(* Logix 5000 Rung export; software revision 16.04 *)

MODULES
   Local : vendor None type None code None
   MVI56E_AFC : vendor None type None code None
END_MODULES

TYPE AFCEProveProcess :   // Prove process output from processor to the module
STRUCT
   Sequencing : AFCEProveSequencing;   // Prover sequencing
   Temperature : REAL;   // Temperature for Single Probe provers. And Inlet Temperature for Dual Probe Provers.
   OutletTemperature : REAL;   // Outlet Temperature for Provers with Dual Probes.
   SwitchBarTemperature : REAL;   // Switch bar temperature
   Pressure : REAL;   // Pressure for Single Probe provers. And Inlet Pressure for Dual Probe Provers.
   OutletPressure : REAL;   // Outlet Pressure for Provers with Dual Probes.
   ProverDensity : REAL;   // Prover density
END_STRUCT
END_TYPE

TYPE AFCEModbusMasterDataType :   // Modbus master data type
STRUCT
   Bit : BOOL;   // bit type
   Word : BOOL;   // word type (16-bit)
   Long : BOOL;   // long integer (32-bit)
   LongRemote : BOOL;   // long integer (32-bit)
END_STRUCT
END_TYPE

TYPE AFCEProveSequencing :   // AFC prove sequencing tag for phase selection and ball positioning
STRUCT
   Phase : AFCEProvePhaseBitmap;   // AFC phase sequencing
   BallPositionReady : BOOL;   // Ball position: Ready (Udir & Bdir only; fwd leg Bdir)
   BallPositionSealed : BOOL;   // Ball position: Sealed (Udir & Bdir only; fwd leg Bdir)
   BallPositionReadyBwdLeg : BOOL;   // Ball position: Ready bwd leg (Bdir only)
   BallPositionSealedBwdLeg : BOOL;   // Ball position: Sealed bwd leg (Bdir only)
END_STRUCT
END_TYPE

TYPE AFCEUtil :   // Used for internal ladder logic usage. These values must not be changed by user application.
STRUCT
   Flags : AFCEFlag;   // Wallclock update commands
   CycleCounter : INT;   // Reflects current block ID calculated by ladder to be sent to the module
   Buffer : AFCEUtilBuffer;
   Block : AFCEUtilBlock;
END_STRUCT
END_TYPE

TYPE AFCEModbusGatewayCommand :   // Modbus Gateway Command
STRUCT
   Config : AFCEModbusGatewayConfig;   // Config data to be entered by the user.
   Trigger : BOOL;   // Trigger the Command, when cleared module has responded.
   Data : INT[200];   // Contains modbus data written to the module (write commands)
END_STRUCT
END_TYPE

TYPE AFCEProveRunResults :   // Run results of the prove. Copied from the module to the pocessor
STRUCT
   CountAttempted : INT;   // Run count attempted
   CountCompleted : INT;   // Run count completed
   CountSelected : INT;   // Run count selected
   RunsSelected : INT;   // Bit Mapped Runs selected for calculations from completed runs
   NewMeterFactor : REAL;   // New meter factor
   ChangeInMeterFactor : REAL;   // Change in meter factor
END_STRUCT
END_TYPE

TYPE AFCEModbusMasterSwap :   // Modbus master swap words/ swap bytes
STRUCT
   SwapWords : BOOL;   // Swap words
   SwapBytes : BOOL;   // Swap bytes
END_STRUCT
END_TYPE

TYPE AFCEModbusMaster :   // Modbus Master. Port 3 must be configured as modbus master through AFC Manager to use this feature.
STRUCT
   Enable : BOOL;   // Enable the modbus master funcionality
   CommandIndex : INT;   // Selects which command index will be executed
   Command : AFCEModbusMasterCommand[10];   // Each command contains a specific modbus request to be sent out of the port
END_STRUCT
END_TYPE

TYPE AFCEFlag :   // Flags contains status information updated by ladder and also trigger bits for clock update
STRUCT
   AFCStopped : BOOL;   // Indicates that the module has sent a new input block to be processed by ladder - UPDATED BY LADDER
   AFCInputSequenceNum : INT;   // Meter number (0 -15) associated to blocks 1-16. Used to update "Profile" (meter type and product group.) UPDATED BY LADDER
END_STRUCT
END_TYPE

TYPE AFCEModbusPassThruBitData :   // AFC Modbus Pass-thru Bit Data
STRUCT
   Data : BOOL[2016];   // Contains received data for bit commands
END_STRUCT
END_TYPE

TYPE AFCEUtilBlockInterrupt :
STRUCT
   Now : BOOL;
   ModbusGateway : DINT;
   EnableDisable : BOOL;
   Analysis : DINT;
END_STRUCT
END_TYPE

TYPE AFCEFirmwareVersion :
STRUCT
   Major : SINT;   // Major Version number
   Minor : SINT;   // Minor Version number
   Revision : INT;   // Revision
END_STRUCT
END_TYPE

TYPE AFCEModbusGateway :   // Modbus Gateway
STRUCT
   Command : AFCEModbusGatewayCommand[10];   // Modbus gateway commands - contains setup and modbus data
END_STRUCT
END_TYPE

TYPE AFCEUtilBuffer :   // Buffer
STRUCT
   Input : INT[250];   // Input buffer contains the complete block to be copied from the module
   Output : INT[248];   // Output buffer contains data the complete block to be copied to the module
   Process : INT[240];
   ArchiveDay : INT[98];
   ArchiveHour : INT[98];
   Prove : INT[26];
   Analysis : INT[198];
   MeterEnableDisable : INT[4];
   StreamEnable : INT[48];
   StreamDisable : INT[48];
   StreamSelect : INT[32];
   MeterSignals : INT[32];
   Calibration : INT[36];
END_STRUCT
END_TYPE

TYPE AFCEUtilBlock :
STRUCT
   ProcessInput : INT;
   InterruptPending : AFCEUtilBlockInterrupt;
   InterruptComplete : AFCEUtilBlockInterrupt;
   NonInterruptPending : AFCEUtilBlockNonInterrupt;
   NonInterruptComplete : AFCEUtilBlockNonInterrupt;
END_STRUCT
END_TYPE

TYPE AFCEProve :   // Prove
STRUCT
   Process : AFCEProveProcess;   // Process Variables
   Signals : AFCEProveSignals;   // AFC Prove Signals (triggers the proving update)
   Config : AFCEProveConfig;   // AFC Prove Control (configuration settings)
   PulseCounts : AFCEProvePulseCount;   // Pulse counts to be updated at the end of the run/pass
   ConfigInput : AFCEProveInputConfig;   // AFC prover input configuration
   Status : AFCEProveStatus;   // AFC prover status
   ErrorCode : INT;   // Prove error code
   ProveControlsEcho : INT;   // AFC module Echos the state of the Prove Controls
   RequestedMeterEcho : INT;   // AFC module Echos the Meter number requested
   RequestedCurvePointEcho : INT;   // AFC module Echos the requested Curve Point
   RunResults : AFCEProveRunResults;   // Prove and run results
   ProveEnabled : BOOL;   // ON if prove is enabled. This flag is coped from inputbuffer[247]
END_STRUCT
END_TYPE

TYPE AFCEProveConfig :   // Controls (configuration settings) associated to the prover
STRUCT
   Enable : AFCEProveConfigEnable;   // Controls at enable
   Accept : AFCEProveConfigAccept;   // Controls at accept
END_STRUCT
END_TYPE

TYPE AFCEWallclock :
STRUCT
   GetAFCTime : BOOL;   // Get current AFC Time
   SetAFCTimeFromPLCTime : BOOL;   // Set AFC time from PLC time. Updates current AFC time
   EnableLocalDateTime : BOOL;   // Enable Local Date Time.
   AFCTime : AFCETime;   // Coordinated Universal Time. Updated by either getting or setting AFC time.
END_STRUCT
END_TYPE

TYPE AFCEModbusMasterConfig :   // Modbus master command settings
STRUCT
   Enable : BOOL;   // Set to 1 to enable command (0=disable)
   FunctionType : BOOL;   // Set to 1 to select write command (0=read command)
   RegisterBank : BOOL;   // Set to 1 to select input register (0=holding register)
   DataType : AFCEModbusMasterDataType;   // Select data type format
   SwapOption : AFCEModbusMasterSwap;   // Select byte and word swap (1 = swap, 0 = no swap)
   TypeSwap : INT;   // This value is calculated by ladder logic and must not be modified by user
   SlaveAddress : INT;   // Modbus slave address of remote device
   ModbusAddress : INT;   // Modbus data address on remote slave
   ElementCount : INT;   // Number of data elements (125 words)
   TransactionID : INT;   // Transaction ID. This value is returned to the ReturnedTransaction ID when the response has been received.
END_STRUCT
END_TYPE

TYPE AFCESiteStatus :   // Site status bits - contains general information about the module - not meter specific
STRUCT
   AFCActive : BOOL;   // AFC active
   ChecksumAlarms : BOOL;   // Checkum alarm active
   Reserved2 : BOOL;
   Reserved3 : BOOL;
   PLCHalted : BOOL;   // PLC in program mode or missing
   CfgChanged : BOOL;   // Configuration changed
   Powerup : BOOL;   // Module powered up
   ColdStart : BOOL;   // Module performed cold start (BBRAM initialized)
   ModbusMasterPending : BOOL;   // Modbus Master Poll Pending
   ModbusMasterComplete : BOOL;   // Modbus Master Poll Complete
   ModbusPassThruPending : BOOL;   // Modbus Pass-thru Input Pending
   CalibrationRequest : BOOL;   // Calibration request from module
   ProverEnabled : BOOL;   // Prover Enabled
   Reserved13 : BOOL;
   Reserved14 : BOOL;
   Reserved15 : BOOL;
END_STRUCT
END_TYPE

TYPE AFCEModuleDef :   // Main user defined data type
STRUCT
   ModbusGateway : AFCEModbusGateway;   // Reads and write data between processor and module modbus table
   ModbusMaster : AFCEModbusMaster;   // Setup modbus master commands to be sent to remote slaves (through Port 3)
   ModbusPassThru : AFCEModbusPassThru;   // Modbus pass-thru data
   SiteStatus : AFCESiteStatus;   // Site status
   MeterAlarms : AFCESiteAlarms;   // Meter Alarms
   Prove : AFCEProve;   // Prover
   Wallclock : AFCEWallclock;   // Set clock and get clock information
   Firmware : AFCEFirmwareVersion;   // Firmware information
   Util : AFCEUtil;   // Used by ladder logic
END_STRUCT
END_TYPE

TYPE AFCEModbusGatewayConfig :   // Modbus Ggateway Configuration
STRUCT
   Enable : BOOL;   // Set to 1 to enable modbus gateway command (0=disable)
   StartRegister : DINT;   // Start modbus address
   RegisterCount : INT;   // Word count (200 max)
   FunctionType : BOOL;   // 0 = read command, 1 = write command
   RegisterType : BOOL;   // 0 = holding register, 1 = input register
   SlaveType : BOOL;   // 0 = primary slave, 1 = virtual slave
END_STRUCT
END_TYPE

TYPE AFCEUtilBlockNonInterrupt :
STRUCT
   Now : BOOL;
   ModbusMasterCommand : BOOL;
   ModbusMasterResponse : BOOL;
   Archive : DINT;
   Prover : BOOL;
   PassThru : BOOL;
   Calibration : BOOL;
END_STRUCT
END_TYPE

TYPE AFCEProveConfigAccept :   // Prove controls at accept. If auto-accept is selected must be available at enable
STRUCT
   RequestedInterpolationPoint : INT;   // Requested interpolation point (0 nearest)
   ApplyMFChangeAllStreams : BOOL;   // Apply change in meter factor to all streams
   ApplyMFChangeCurve : BOOL;   // Apply change in meter factor to all curve points
   ApplyNewMF : BOOL;   // CApply new meter factor
END_STRUCT
END_TYPE

TYPE AFCEProvePhaseBitmap :   // AFC prove phase bitmap
STRUCT
   NotSelected : BOOL;   // Not selected
   Active : BOOL;   // Active, not counting
   CountingPast1stSwitch : BOOL;   // Counting past 1st switch for Udir and forward leg for Bdir)
   Past2ndSwitchFwdLeg : BOOL;   // Past 2nd switch forward leg (bidirectional only)
   Past1stSwithRetLeg : BOOL;   // Past 1st switch return leg (bidirectional only)
   RunComplete : BOOL;   // Run complete. past 2nd switch.
END_STRUCT
END_TYPE

TYPE AFCETime :   // AFC time format used for wallclock update.
STRUCT
   Year : DINT;   // Year
   Month : DINT;   // Month
   Day : DINT;   // Day
   Hour : DINT;   // Hour
   Minute : DINT;   // Minute
   second : DINT;   // Seconds
END_STRUCT
END_TYPE

TYPE AFCEProveSignals :   // Contains the proving signals that will trigger specific tasks from the module
STRUCT
   EnableProve : BOOL;   // Enables the prove
   AcceptProve : BOOL;   // Accepts the prove
   RejectProve : BOOL;   // Reject the prove
   RunStart : BOOL;   // Starts the run
   RunComplete : BOOL;   // Flags that the run is complete
   RunCancel : BOOL;   // Cancels the run
   RunDelete : BOOL;   // Deletes the run
   PassComplete : BOOL;   // Flag that the pass is complete
   PauseProve : BOOL;   // Pauses the Proving Process
   AbortProve : BOOL;   // Aborts the prove
END_STRUCT
END_TYPE

TYPE AFCEModbusPassThru :   // AFC Modbus Pass-thru
STRUCT
   Enable : BOOL;   // Set to 1 to enable pass-thru functionality (requires AFC Manager setting)
   MessagePresent : BOOL;   // Message present in the response block
   GetMessage : BOOL;   // Get the pass-thru message. When the bit is cleared the message has been transferred to the PLC.
   FunctionBitWrite : BOOL;   // Function bit write
   OverflowError : BOOL;   // Overflow error flag
   ModbusAddress : INT;   // Destination modbus address
   RegisterCount : INT;   // Number of elements associated to command
   ReadDataWord : INT[125];   // Contains received data for word commands
   ReadDataBit : AFCEModbusPassThruBitData;   // Contains received data for bit commands
END_STRUCT
END_TYPE

TYPE AFCEProveInputConfig :   // Prove input block results - prover configuration
STRUCT
   Type : INT;   // Prover type
   Options : INT;   // Prover options
   RunsPerProveTotal : INT;   // Total runs per prove
   RunsPerProveSelected : INT;   // Selected runs per prove
   MaxRunsBeforeAbort : INT;   // Max total runs before abort
   ShortPassesPerRun : INT;   // Short passes per run if bidir = 2 , else 0
END_STRUCT
END_TYPE

TYPE AFCEProveStatus :   // Status of the prove (returned from the module to the processor)
STRUCT
   ProveAccepted : BOOL;   // Prove was accepted
   MeterFactorApplied : BOOL;   // Meter factor was applied
   MFAppliedToCurve : BOOL;   // Meter factor was applied to all points in the curve
   MFAppliedToStreams : BOOL;   // Meter factor was applied to all streams
   ProveRejectedByCommand : BOOL;   // Prove was rejected by command
   ProveRejectedNoRuns : BOOL;   // Prove was rejected - empty prove (no runs)
   ProveRejectedDivideBy0 : BOOL;   // Prove was rejected - divide by 0
   ProveEnabled : BOOL;   // Prove is enabled
   ProvingRunInProgress : BOOL;   // Proving run is in progress
   ProveRejectedAbort : BOOL;   // Prove rejected: abort
   ProvePaused : BOOL;   // Prove is paused
   RunCancelled : BOOL;   // Run Is cancelled
   RunTimedOut : BOOL;   // Run timed out
END_STRUCT
END_TYPE

TYPE AFCEProveConfigEnable :   // Prove controls at enable
STRUCT
   MeterNumber : INT;   // Meter number requested (1-16)
   AutoAcceptProve : BOOL;   // Auto-accept the prove
   AutoContinueProve : BOOL;   // Auto-continue the prove
END_STRUCT
END_TYPE

TYPE AFCEModbusMasterCommand :   // Modbus Master Command
STRUCT
   Config : AFCEModbusMasterConfig;   // Modbus Master Configuration
   ErrorCode : INT;   // Error Code associated to Modbus Master Command
   Pending : BOOL;   // Pending Modbus Master Command - waiting for Modbus Response
   ReturnedTransactionID : DINT;   // Changes to Config.TransactionID value when response has returned.
   Data : INT[100];   // Read or Write Data
END_STRUCT
END_TYPE

TYPE AFCEProvePulseCount :   // Values to be supplied at the end of the pass/run
STRUCT
   Meter : DINT;   // Meter pulse count
   MasterMeter : DINT;   // Master meter pulse count
END_STRUCT
END_TYPE

TYPE AFCESiteAlarms :   // Indicates if a meter has any alarms
STRUCT
   Meter1 : BOOL;   // Meter in alarm
   Meter2 : BOOL;   // Meter in alarm
   Meter3 : BOOL;   // Meter in alarm
   Meter4 : BOOL;   // Meter in alarm
   Meter5 : BOOL;   // Meter in alarm
   Meter6 : BOOL;   // Meter in alarm
   Meter7 : BOOL;   // Meter in alarm
   Meter8 : BOOL;   // Meter in alarm
   Meter9 : BOOL;   // Meter in alarm
   Meter10 : BOOL;   // Meter in alarm
   Meter11 : BOOL;   // Meter in alarm
   Meter12 : BOOL;   // Meter in alarm
   Meter13 : BOOL;   // Meter in alarm
   Meter14 : BOOL;   // Meter in alarm
   Meter15 : BOOL;   // Meter in alarm
   Meter16 : BOOL;   // Meter in alarm
END_STRUCT
END_TYPE

ADD_ON_INSTRUCTION AOI56EAFC   (* revision 2.6, vendor ProSoft Technology Inc., ExecutePrescan *)
// Add-On instruction for the MVI56E-AFC.
// Module Interface.
// Revision note:
// Modified Move Instruction Source Value from 7 to 10 in Rung 18 to pull Firmware Rev Block.
// Help:
// Compatible with version 4.01 of MVI56E-AFC firmware or higher.
// v2.2 Add PLC Mediation. Period task, wall clock and MB passthru fix.
// v2.4 Ability to set UTC or local date time from ladder.
// v2.5: Made changes to the ModbusGatewayConfig UDT StartRegister Tag Data Type from INT to DINT.
// v2.6: Modified Move Instruction Source Value from 7 to 10 in Rung 18 to pull Firmware Rev Block.
VAR_IN_OUT
   ConnectionInput : INT[250]; {required}
   ConnectionOutput : INT[248]; {required}
   AFC : AFCEModuleDef; {required}
        .UTIL.BUFFER.PROVE[12]   // Main user defined data type Buffer
END_VAR
VAR
   WallclockCurrentPLCTime : DINT[7];
   UTCTimeDelta : DINT;
   TimeZoneString : STRING;
   StoppedTimer : TIMER;
   ProverSignals : DINT;
   ProverPhase : DINT;
   ProverControls : DINT;
   ProveEnabled : BOOL;
   ProfileBlockID : DINT;
   Offset1 : DINT;
   NotStoppedTimer : TIMER;
   ModbusPassThruOverflowError : BOOL;
   ModbusPassThruOutput : DINT;
   ModbusPassThruMessagePresent : BOOL;
   ModbusPassThruFunctionBitWrite : BOOL;
   ModbusMasterTransactionNumber : DINT;
   ModbusMasterReadWrite : BOOL;   // 0=Read 1=Write
   ModbusMasterPending : BOOL;
   ModbusMasterOutput : INT;
   CycleCounterPreviousStopped : INT;
   ModbusMasterLongCount : DINT;
   ModbusGatewayReadWrite : BOOL;   // 0=Read, 1=Write
   ModbusGatewayOutput : DINT;
   ModbusGatewayIndexBitPosition : DINT;
   ModbusGatewayIndex : DINT;
   MJFAULTS : DINT[12];
   LocalHourChange : DINT;
   LatchStopped : BOOL;
   ForceReset : BOOL;
   AvoidBufferOverflowFault : DINT;   // Need this to prevent Overflow Minor Fault
   AFCTime : AFCETime;
END_VAR

ROUTINE Logic   (* ladder *)
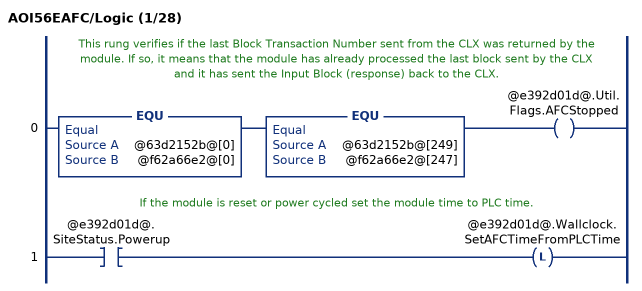
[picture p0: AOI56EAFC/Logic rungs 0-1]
   // This rung verifies if the last Block Transaction Number sent from the CLX was returned by the module. If so, it means that the module has already processed the last block sent by the CLX and it has sent the Input Block (response) back to the CLX.
   0: EQU(@63d2152b@[0],@f62a66e2@[0])EQU(@63d2152b@[249],@f62a66e2@[247])OTE(@e392d01d@.Util.Flags.AFCStopped);
   // If the module is reset or power cycled set the module time to PLC time.
   1: XIC(@e392d01d@.SiteStatus.Powerup)OTL(@e392d01d@.Wallclock.SetAFCTimeFromPLCTime);
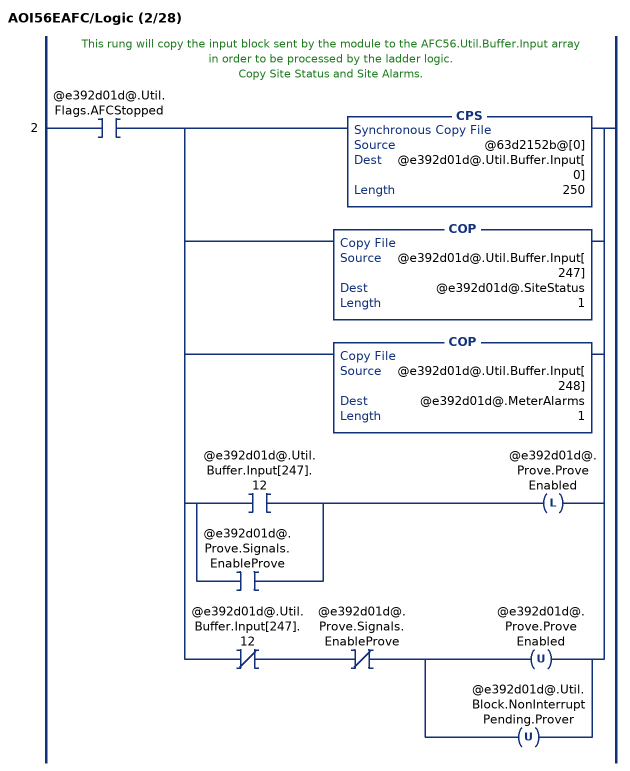
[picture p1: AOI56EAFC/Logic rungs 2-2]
   // This rung will copy the input block sent by the module to the AFC56.Util.Buffer.Input array in order to be processed by the ladder logic.
   // Copy Site Status and Site Alarms.
   2: XIC(@e392d01d@.Util.Flags.AFCStopped)[CPS(@63d2152b@[0],@e392d01d@.Util.Buffer.Input[0],250) ,COP(@e392d01d@.Util.Buffer.Input[247],@e392d01d@.SiteStatus,1) ,COP(@e392d01d@.Util.Buffer.Input[248],@e392d01d@.MeterAlarms,1) ,[XIC(@e392d01d@.Util.Buffer.Input[247].12) ,XIC(@e392d01d@.Prove.Signals.EnableProve) ] OTL(@e392d01d@.Prove.ProveEnabled) ,XIO(@e392d01d@.Util.Buffer.Input[247].12) XIO(@e392d01d@.Prove.Signals.EnableProve) [OTU(@e392d01d@.Prove.ProveEnabled) ,OTU(@e392d01d@.Util.Block.NonInterruptPending.Prover) ] ];
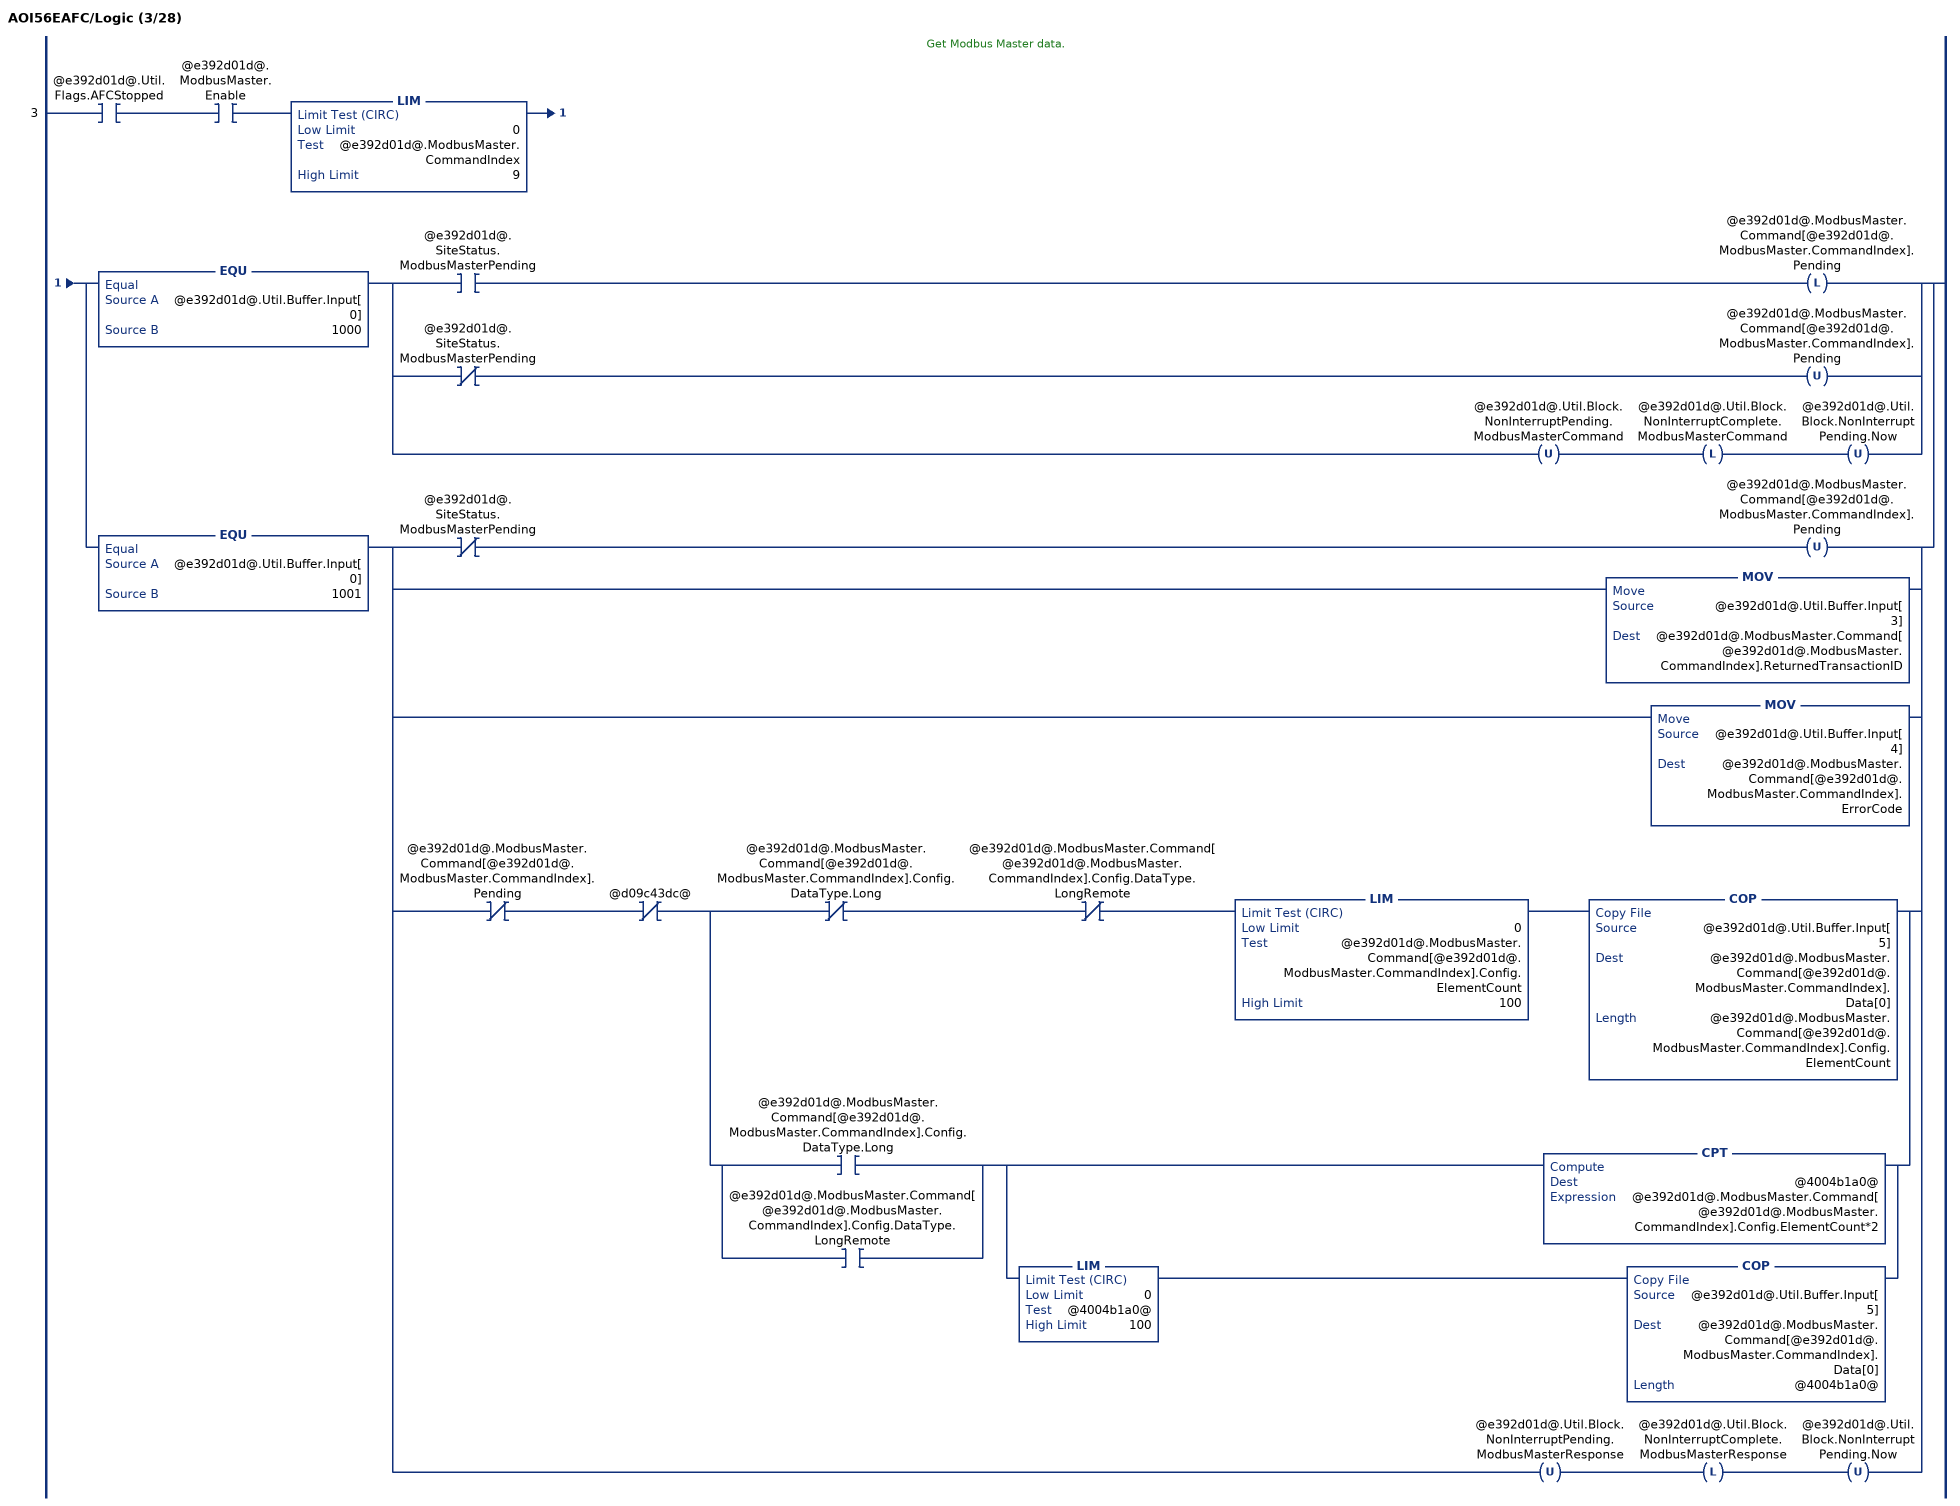
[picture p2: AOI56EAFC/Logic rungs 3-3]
   // Get Modbus Master data.
   3: XIC(@e392d01d@.Util.Flags.AFCStopped)XIC(@e392d01d@.ModbusMaster.Enable)LIM(0,@e392d01d@.ModbusMaster.CommandIndex,9)[EQU(@e392d01d@.Util.Buffer.Input[0],1000) [XIC(@e392d01d@.SiteStatus.ModbusMasterPending) OTL(@e392d01d@.ModbusMaster.Command[@e392d01d@.ModbusMaster.CommandIndex].Pending) ,XIO(@e392d01d@.SiteStatus.ModbusMasterPending) OTU(@e392d01d@.ModbusMaster.Command[@e392d01d@.ModbusMaster.CommandIndex].Pending) ,OTU(@e392d01d@.Util.Block.NonInterruptPending.ModbusMasterCommand) OTL(@e392d01d@.Util.Block.NonInterruptComplete.ModbusMasterCommand) OTU(@e392d01d@.Util.Block.NonInterruptPending.Now) ] ,EQU(@e392d01d@.Util.Buffer.Input[0],1001) [XIO(@e392d01d@.SiteStatus.ModbusMasterPending) OTU(@e392d01d@.ModbusMaster.Command[@e392d01d@.ModbusMaster.CommandIndex].Pending) ,MOV(@e392d01d@.Util.Buffer.Input[3],@e392d01d@.ModbusMaster.Command[@e392d01d@.ModbusMaster.CommandIndex].ReturnedTransactionID) ,MOV(@e392d01d@.Util.Buffer.Input[4],@e392d01d@.ModbusMaster.Command[@e392d01d@.ModbusMaster.CommandIndex].ErrorCode) ,XIO(@e392d01d@.ModbusMaster.Command[@e392d01d@.ModbusMaster.CommandIndex].Pending) XIO(@d09c43dc@) [XIO(@e392d01d@.ModbusMaster.Command[@e392d01d@.ModbusMaster.CommandIndex].Config.DataType.Long) XIO(@e392d01d@.ModbusMaster.Command[@e392d01d@.ModbusMaster.CommandIndex].Config.DataType.LongRemote) LIM(0,@e392d01d@.ModbusMaster.Command[@e392d01d@.ModbusMaster.CommandIndex].Config.ElementCount,100) COP(@e392d01d@.Util.Buffer.Input[5],@e392d01d@.ModbusMaster.Command[@e392d01d@.ModbusMaster.CommandIndex].Data[0],@e392d01d@.ModbusMaster.Command[@e392d01d@.ModbusMaster.CommandIndex].Config.ElementCount) ,[XIC(@e392d01d@.ModbusMaster.Command[@e392d01d@.ModbusMaster.CommandIndex].Config.DataType.Long) ,XIC(@e392d01d@.ModbusMaster.Command[@e392d01d@.ModbusMaster.CommandIndex].Config.DataType.LongRemote) ] [CPT(@4004b1a0@,@e392d01d@.ModbusMaster.Command[@e392d01d@.ModbusMaster.CommandIndex].Config.ElementCount*2) ,LIM(0,@4004b1a0@,100) COP(@e392d01d@.Util.Buffer.Input[5],@e392d01d@.ModbusMaster.Command[@e392d01d@.ModbusMaster.CommandIndex].Data[0],@4004b1a0@) ] ] ,OTU(@e392d01d@.Util.Block.NonInterruptPending.ModbusMasterResponse) OTL(@e392d01d@.Util.Block.NonInterruptComplete.ModbusMasterResponse) OTU(@e392d01d@.Util.Block.NonInterruptPending.Now) ] ];
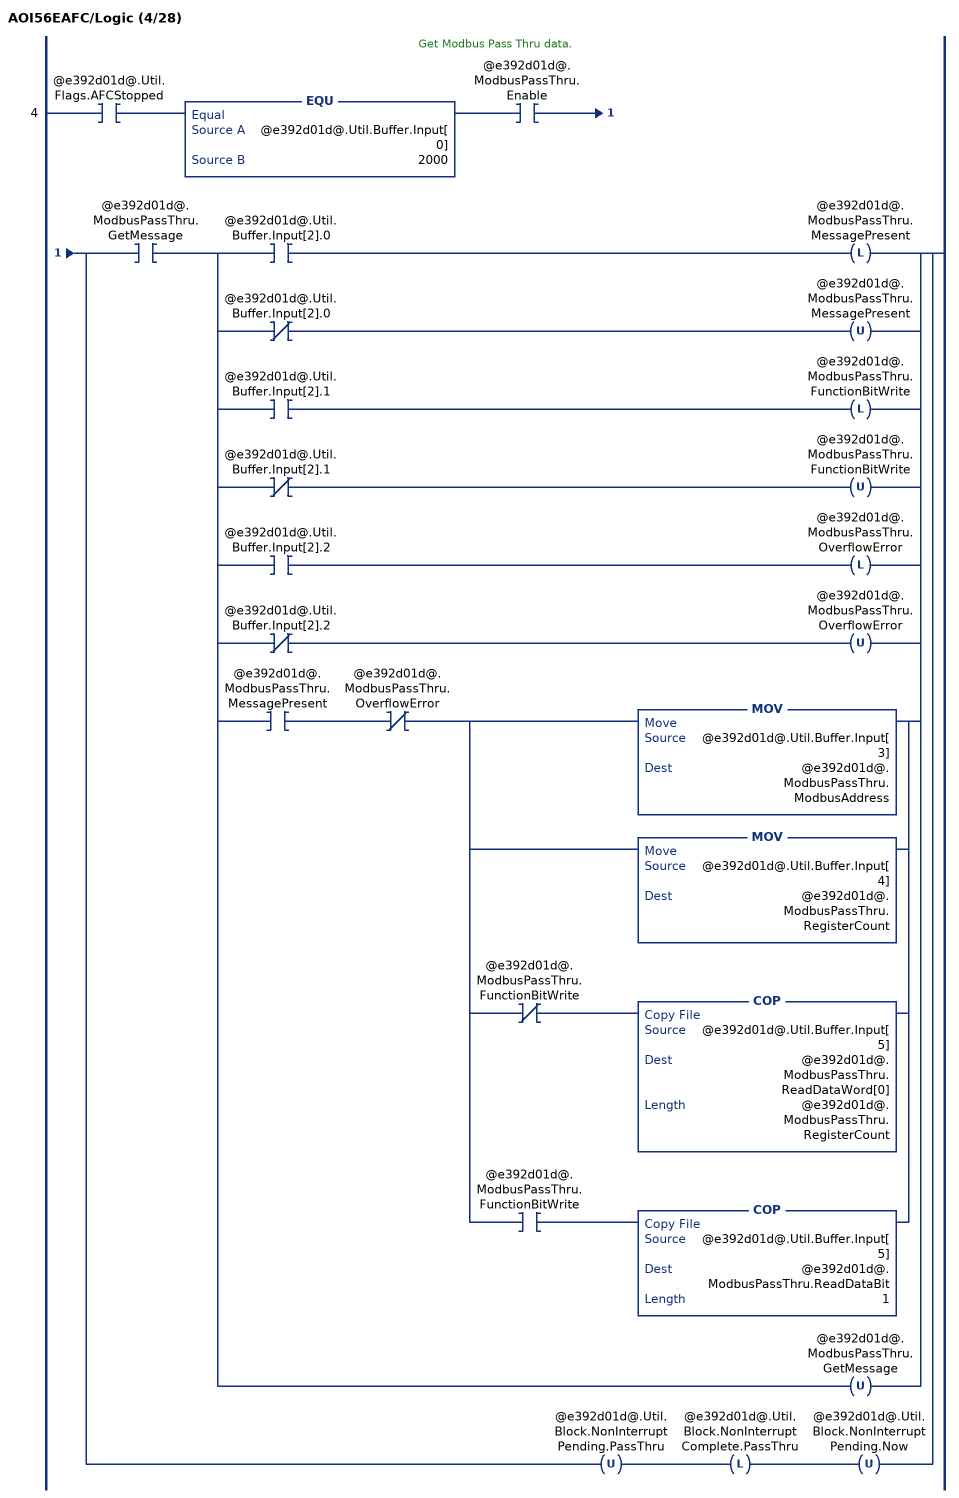
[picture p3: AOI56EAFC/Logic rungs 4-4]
   // Get Modbus Pass Thru data.
   4: XIC(@e392d01d@.Util.Flags.AFCStopped)EQU(@e392d01d@.Util.Buffer.Input[0],2000)XIC(@e392d01d@.ModbusPassThru.Enable)[XIC(@e392d01d@.ModbusPassThru.GetMessage) [[XIC(@e392d01d@.Util.Buffer.Input[2].0) OTL(@e392d01d@.ModbusPassThru.MessagePresent) ,XIO(@e392d01d@.Util.Buffer.Input[2].0) OTU(@e392d01d@.ModbusPassThru.MessagePresent) ,XIC(@e392d01d@.Util.Buffer.Input[2].1) OTL(@e392d01d@.ModbusPassThru.FunctionBitWrite) ,XIO(@e392d01d@.Util.Buffer.Input[2].1) OTU(@e392d01d@.ModbusPassThru.FunctionBitWrite) ,XIC(@e392d01d@.Util.Buffer.Input[2].2) OTL(@e392d01d@.ModbusPassThru.OverflowError) ,XIO(@e392d01d@.Util.Buffer.Input[2].2) OTU(@e392d01d@.ModbusPassThru.OverflowError) ] ,XIC(@e392d01d@.ModbusPassThru.MessagePresent) XIO(@e392d01d@.ModbusPassThru.OverflowError) [MOV(@e392d01d@.Util.Buffer.Input[3],@e392d01d@.ModbusPassThru.ModbusAddress) ,MOV(@e392d01d@.Util.Buffer.Input[4],@e392d01d@.ModbusPassThru.RegisterCount) ,XIO(@e392d01d@.ModbusPassThru.FunctionBitWrite) COP(@e392d01d@.Util.Buffer.Input[5],@e392d01d@.ModbusPassThru.ReadDataWord[0],@e392d01d@.ModbusPassThru.RegisterCount) ,XIC(@e392d01d@.ModbusPassThru.FunctionBitWrite) COP(@e392d01d@.Util.Buffer.Input[5],@e392d01d@.ModbusPassThru.ReadDataBit,1) ] ,OTU(@e392d01d@.ModbusPassThru.GetMessage) ] ,OTU(@e392d01d@.Util.Block.NonInterruptPending.PassThru) OTL(@e392d01d@.Util.Block.NonInterruptComplete.PassThru) OTU(@e392d01d@.Util.Block.NonInterruptPending.Now) ];
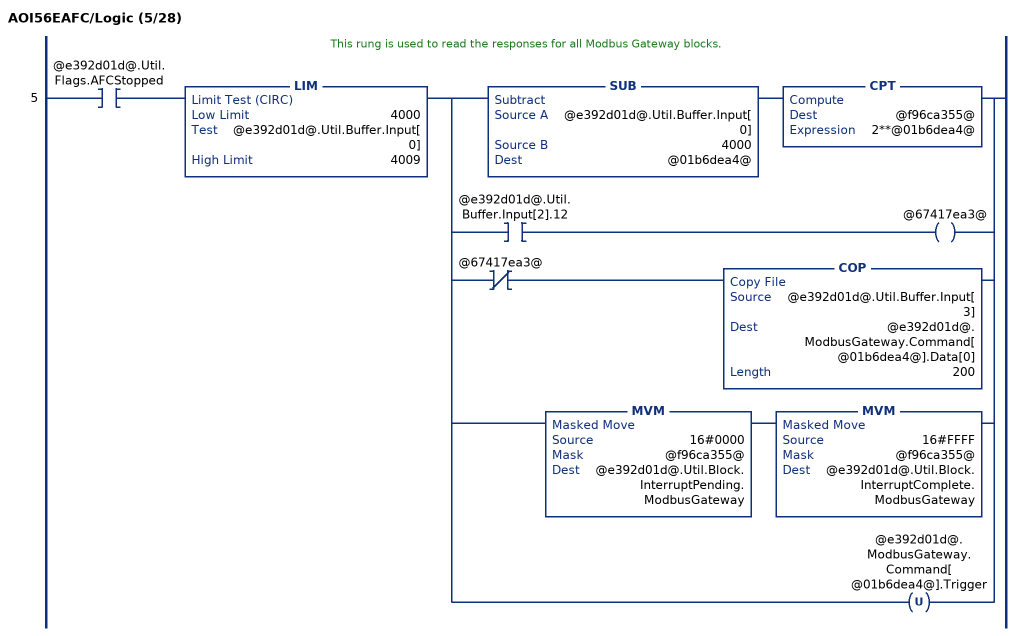
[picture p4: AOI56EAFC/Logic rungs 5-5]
   // This rung is used to read the responses for all Modbus Gateway blocks.
   5: XIC(@e392d01d@.Util.Flags.AFCStopped)LIM(4000,@e392d01d@.Util.Buffer.Input[0],4009)[SUB(@e392d01d@.Util.Buffer.Input[0],4000,@01b6dea4@) CPT(@f96ca355@,2**@01b6dea4@) ,XIC(@e392d01d@.Util.Buffer.Input[2].12) OTE(@67417ea3@) ,XIO(@67417ea3@) COP(@e392d01d@.Util.Buffer.Input[3],@e392d01d@.ModbusGateway.Command[@01b6dea4@].Data[0],200) ,MVM(16#0000,@f96ca355@,@e392d01d@.Util.Block.InterruptPending.ModbusGateway) MVM(16#FFFF,@f96ca355@,@e392d01d@.Util.Block.InterruptComplete.ModbusGateway) ,OTU(@e392d01d@.ModbusGateway.Command[@01b6dea4@].Trigger) ];
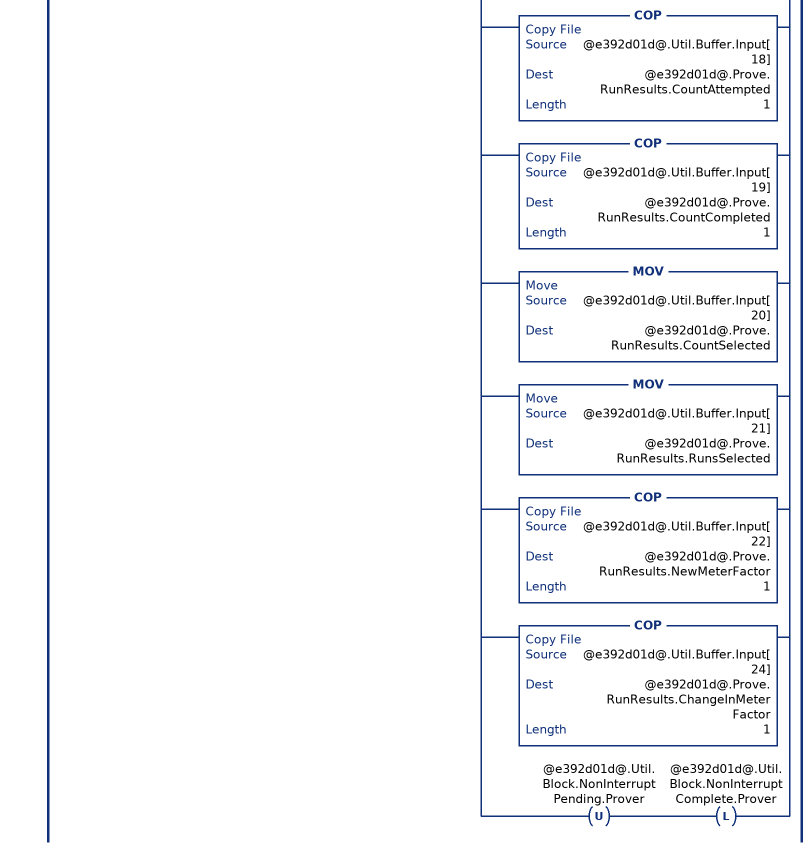
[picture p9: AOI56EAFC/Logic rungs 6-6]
   6: XIC(@e392d01d@.Util.Flags.AFCStopped)EQU(@e392d01d@.Util.Buffer.Input[0],5000)[XIC(@1f384e10@.1) OTU(@e392d01d@.Prove.Signals.EnableProve) ,XIC(@1f384e10@.2) OTU(@e392d01d@.Prove.Signals.AcceptProve) ,XIC(@1f384e10@.3) OTU(@e392d01d@.Prove.Signals.RejectProve) ,XIC(@1f384e10@.4) OTU(@e392d01d@.Prove.Signals.RunStart) ,XIC(@1f384e10@.5) OTU(@e392d01d@.Prove.Signals.RunComplete) ,XIC(@1f384e10@.6) OTU(@e392d01d@.Prove.Signals.RunCancel) ,XIC(@1f384e10@.7) OTU(@e392d01d@.Prove.Signals.RunDelete) ,XIC(@1f384e10@.9) OTU(@e392d01d@.Prove.Signals.PassComplete) ,XIC(@1f384e10@.12) OTU(@e392d01d@.Prove.Signals.PauseProve) ,XIC(@1f384e10@.14) OTU(@e392d01d@.Prove.Signals.AbortProve) ,MOV(@e392d01d@.Util.Buffer.Input[3],@e392d01d@.Prove.ConfigInput.Type) ,MOV(@e392d01d@.Util.Buffer.Input[4],@e392d01d@.Prove.ConfigInput.Options) ,MOV(@e392d01d@.Util.Buffer.Input[5],@e392d01d@.Prove.ConfigInput.RunsPerProveTotal) ,MOV(@e392d01d@.Util.Buffer.Input[6],@e392d01d@.Prove.ConfigInput.RunsPerProveSelected) ,MOV(@e392d01d@.Util.Buffer.Input[7],@e392d01d@.Prove.ConfigInput.MaxRunsBeforeAbort) ,MOV(@e392d01d@.Util.Buffer.Input[8],@e392d01d@.Prove.ConfigInput.ShortPassesPerRun) ,XIC(@e392d01d@.Util.Buffer.Input[12].0) OTL(@e392d01d@.Prove.Status.ProveAccepted) ,XIO(@e392d01d@.Util.Buffer.Input[12].0) OTU(@e392d01d@.Prove.Status.ProveAccepted) ,XIC(@e392d01d@.Util.Buffer.Input[12].1) OTL(@e392d01d@.Prove.Status.MeterFactorApplied) ,XIO(@e392d01d@.Util.Buffer.Input[12].1) OTU(@e392d01d@.Prove.Status.MeterFactorApplied) ,XIC(@e392d01d@.Util.Buffer.Input[12].2) OTL(@e392d01d@.Prove.Status.MFAppliedToCurve) ,XIO(@e392d01d@.Util.Buffer.Input[12].2) OTU(@e392d01d@.Prove.Status.MFAppliedToCurve) ,XIC(@e392d01d@.Util.Buffer.Input[12].3) OTL(@e392d01d@.Prove.Status.MFAppliedToStreams) ,XIO(@e392d01d@.Util.Buffer.Input[12].3) OTU(@e392d01d@.Prove.Status.MFAppliedToStreams) ,XIC(@e392d01d@.Util.Buffer.Input[12].4) OTL(@e392d01d@.Prove.Status.ProveRejectedByCommand) ,XIO(@e392d01d@.Util.Buffer.Input[12].4) OTU(@e392d01d@.Prove.Status.ProveRejectedByCommand) ,XIC(@e392d01d@.Util.Buffer.Input[12].5) OTL(@e392d01d@.Prove.Status.ProveRejectedNoRuns) ,XIO(@e392d01d@.Util.Buffer.Input[12].5) OTU(@e392d01d@.Prove.Status.ProveRejectedNoRuns) ,XIC(@e392d01d@.Util.Buffer.Input[12].6) OTL(@e392d01d@.Prove.Status.ProveRejectedDivideBy0) ,XIO(@e392d01d@.Util.Buffer.Input[12].6) OTU(@e392d01d@.Prove.Status.ProveRejectedDivideBy0) ,XIC(@e392d01d@.Util.Buffer.Input[12].8) OTL(@e392d01d@.Prove.Status.ProveEnabled) ,[XIO(@e392d01d@.Util.Buffer.Input[12].8) ,XIC(@1f384e10@.2) ,XIC(@1f384e10@.3) ,XIC(@1f384e10@.14) ] OTU(@e392d01d@.Prove.Status.ProveEnabled) ,XIC(@e392d01d@.Util.Buffer.Input[12].9) OTL(@e392d01d@.Prove.Status.ProvingRunInProgress) ,XIO(@e392d01d@.Util.Buffer.Input[12].9) OTU(@e392d01d@.Prove.Status.ProvingRunInProgress) ,XIC(@e392d01d@.Util.Buffer.Input[12].10) OTL(@e392d01d@.Prove.Status.ProvePaused) ,XIO(@e392d01d@.Util.Buffer.Input[12].10) OTU(@e392d01d@.Prove.Status.ProvePaused) ,XIC(@e392d01d@.Util.Buffer.Input[12].11) OTL(@e392d01d@.Prove.Status.RunCancelled) ,XIO(@e392d01d@.Util.Buffer.Input[12].11) OTU(@e392d01d@.Prove.Status.RunCancelled) ,XIC(@e392d01d@.Util.Buffer.Input[12].12) OTL(@e392d01d@.Prove.Status.RunTimedOut) ,XIO(@e392d01d@.Util.Buffer.Input[12].12) OTU(@e392d01d@.Prove.Status.RunTimedOut) ,XIC(@e392d01d@.Util.Buffer.Input[12].14) OTL(@e392d01d@.Prove.Status.ProveRejectedAbort) ,XIO(@e392d01d@.Util.Buffer.Input[12].14) OTU(@e392d01d@.Prove.Status.ProveRejectedAbort) ,MOV(@e392d01d@.Util.Buffer.Input[13],@e392d01d@.Prove.ErrorCode) ,MOV(@e392d01d@.Util.Buffer.Input[14],@e392d01d@.Prove.ProveControlsEcho) ,MOV(@e392d01d@.Util.Buffer.Input[15],@e392d01d@.Prove.RequestedMeterEcho) ,MOV(@e392d01d@.Util.Buffer.Input[17],@e392d01d@.Prove.RequestedCurvePointEcho) ,COP(@e392d01d@.Util.Buffer.Input[18],@e392d01d@.Prove.RunResults.CountAttempted,1) ,COP(@e392d01d@.Util.Buffer.Input[19],@e392d01d@.Prove.RunResults.CountCompleted,1) ,MOV(@e392d01d@.Util.Buffer.Input[20],@e392d01d@.Prove.RunResults.CountSelected) ,MOV(@e392d01d@.Util.Buffer.Input[21],@e392d01d@.Prove.RunResults.RunsSelected) ,COP(@e392d01d@.Util.Buffer.Input[22],@e392d01d@.Prove.RunResults.NewMeterFactor,1) ,COP(@e392d01d@.Util.Buffer.Input[24],@e392d01d@.Prove.RunResults.ChangeInMeterFactor,1) ,OTU(@e392d01d@.Util.Block.NonInterruptPending.Prover) OTL(@e392d01d@.Util.Block.NonInterruptComplete.Prover) ];
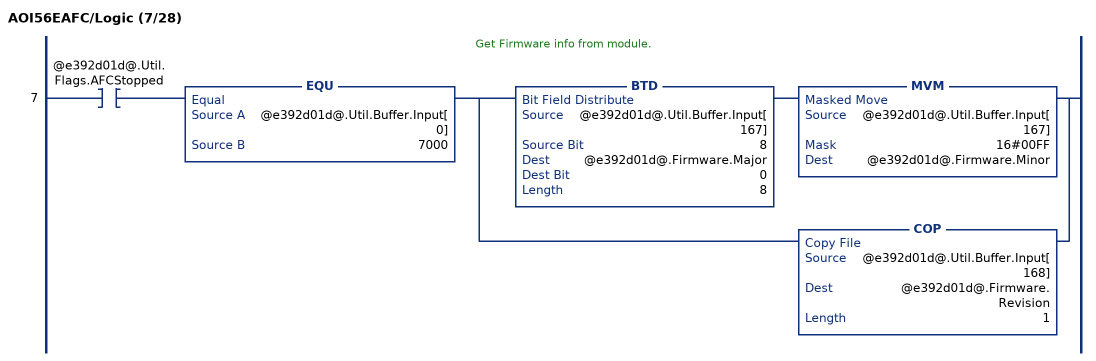
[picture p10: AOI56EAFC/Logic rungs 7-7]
   // Get Firmware info from module.
   7: XIC(@e392d01d@.Util.Flags.AFCStopped)EQU(@e392d01d@.Util.Buffer.Input[0],7000)[BTD(@e392d01d@.Util.Buffer.Input[167],8,@e392d01d@.Firmware.Major,0,8) MVM(@e392d01d@.Util.Buffer.Input[167],16#00FF,@e392d01d@.Firmware.Minor) ,COP(@e392d01d@.Util.Buffer.Input[168],@e392d01d@.Firmware.Revision,1) ];
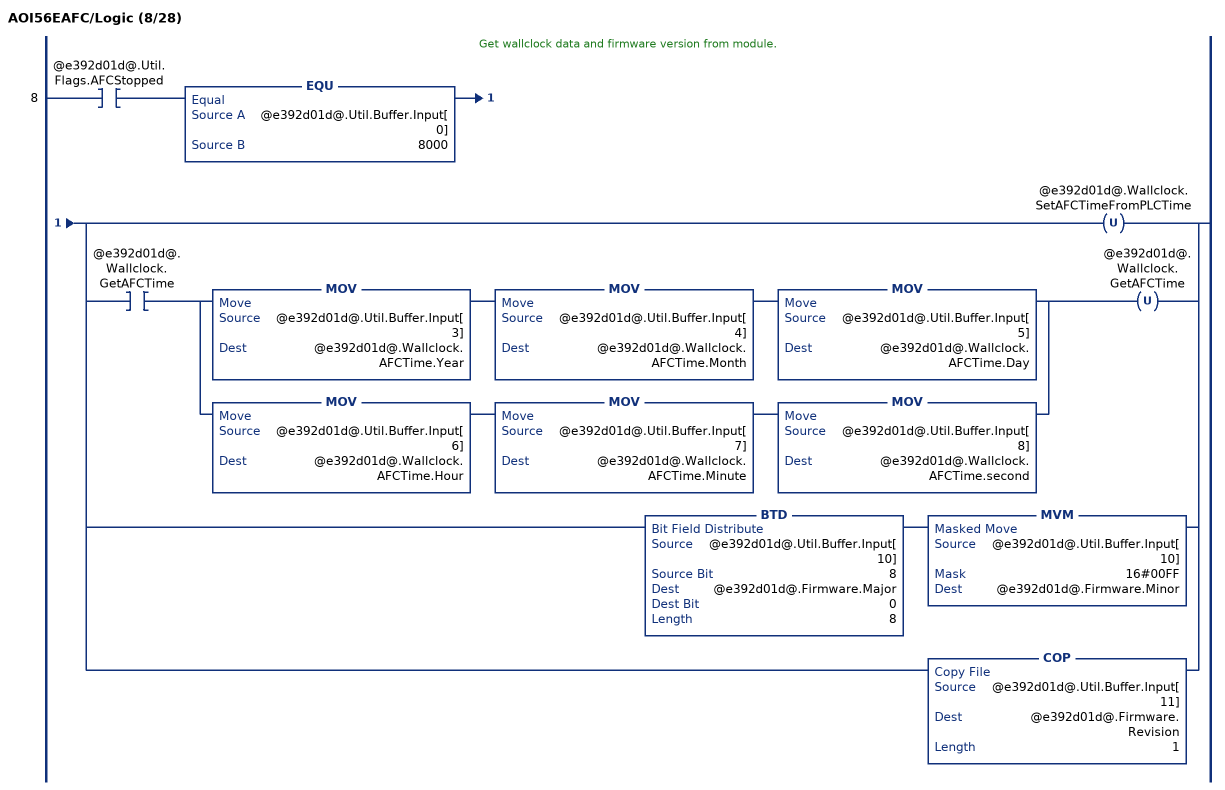
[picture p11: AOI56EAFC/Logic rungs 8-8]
   // Get wallclock data and firmware version from module.
   8: XIC(@e392d01d@.Util.Flags.AFCStopped)EQU(@e392d01d@.Util.Buffer.Input[0],8000)[OTU(@e392d01d@.Wallclock.SetAFCTimeFromPLCTime) ,XIC(@e392d01d@.Wallclock.GetAFCTime) [MOV(@e392d01d@.Util.Buffer.Input[3],@e392d01d@.Wallclock.AFCTime.Year) MOV(@e392d01d@.Util.Buffer.Input[4],@e392d01d@.Wallclock.AFCTime.Month) MOV(@e392d01d@.Util.Buffer.Input[5],@e392d01d@.Wallclock.AFCTime.Day) ,MOV(@e392d01d@.Util.Buffer.Input[6],@e392d01d@.Wallclock.AFCTime.Hour) MOV(@e392d01d@.Util.Buffer.Input[7],@e392d01d@.Wallclock.AFCTime.Minute) MOV(@e392d01d@.Util.Buffer.Input[8],@e392d01d@.Wallclock.AFCTime.second) ] OTU(@e392d01d@.Wallclock.GetAFCTime) ,[BTD(@e392d01d@.Util.Buffer.Input[10],8,@e392d01d@.Firmware.Major,0,8) MVM(@e392d01d@.Util.Buffer.Input[10],16#00FF,@e392d01d@.Firmware.Minor) ,COP(@e392d01d@.Util.Buffer.Input[11],@e392d01d@.Firmware.Revision,1) ] ];
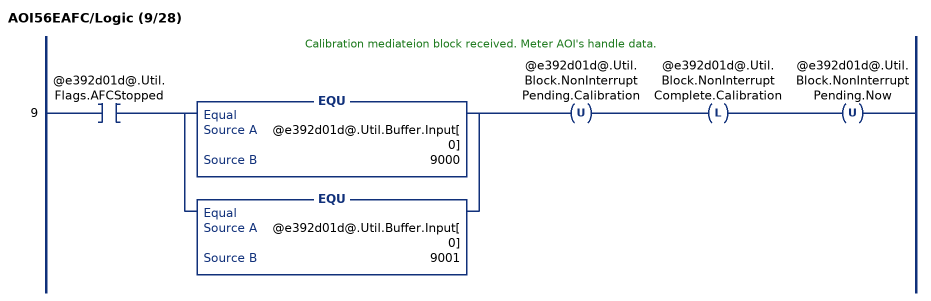
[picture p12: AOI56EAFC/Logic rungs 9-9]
   // Calibration mediateion block received. Meter AOI's handle data.
   9: XIC(@e392d01d@.Util.Flags.AFCStopped)[EQU(@e392d01d@.Util.Buffer.Input[0],9000) ,EQU(@e392d01d@.Util.Buffer.Input[0],9001) ]OTU(@e392d01d@.Util.Block.NonInterruptPending.Calibration)OTL(@e392d01d@.Util.Block.NonInterruptComplete.Calibration)OTU(@e392d01d@.Util.Block.NonInterruptPending.Now);
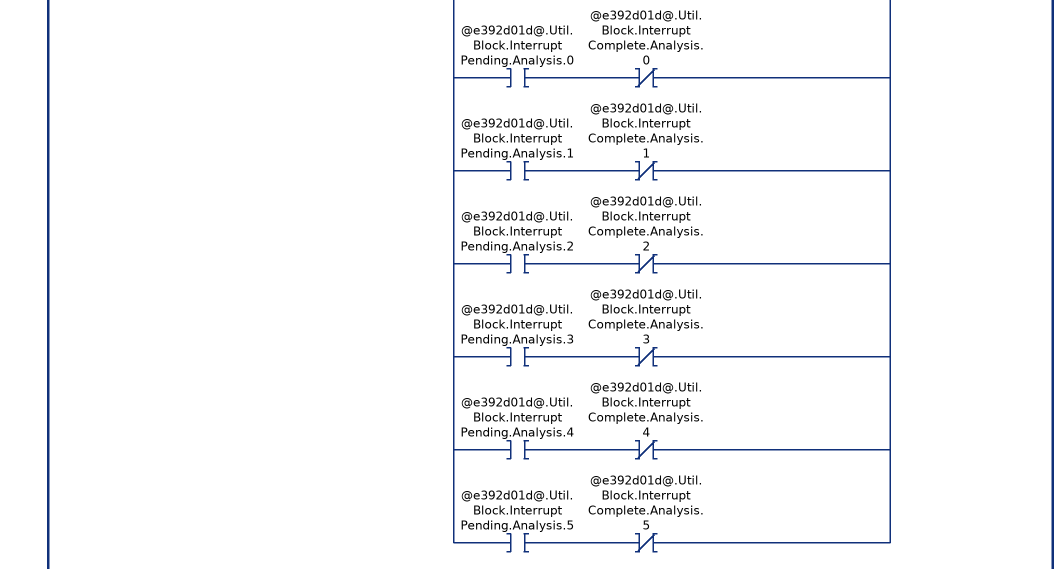
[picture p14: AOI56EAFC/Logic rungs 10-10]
   // Interrupt blocks (3000, 4000 and 7000) are interleaved between Process Input blocks.
   // Check if any interrupt block is pending.
   10: XIC(@e392d01d@.Util.Flags.AFCStopped)LIM(1,@e392d01d@.Util.Buffer.Input[0],15)[XIC(@e392d01d@.ModbusGateway.Command[0].Trigger) XIO(@e392d01d@.Util.Block.InterruptComplete.ModbusGateway.0) OTL(@e392d01d@.Util.Block.InterruptPending.ModbusGateway.0) ,XIC(@e392d01d@.ModbusGateway.Command[1].Trigger) XIO(@e392d01d@.Util.Block.InterruptComplete.ModbusGateway.1) OTL(@e392d01d@.Util.Block.InterruptPending.ModbusGateway.1) ,XIC(@e392d01d@.ModbusGateway.Command[2].Trigger) XIO(@e392d01d@.Util.Block.InterruptComplete.ModbusGateway.2) OTL(@e392d01d@.Util.Block.InterruptPending.ModbusGateway.2) ,XIC(@e392d01d@.ModbusGateway.Command[3].Trigger) XIO(@e392d01d@.Util.Block.InterruptComplete.ModbusGateway.3) OTL(@e392d01d@.Util.Block.InterruptPending.ModbusGateway.3) ,XIC(@e392d01d@.ModbusGateway.Command[4].Trigger) XIO(@e392d01d@.Util.Block.InterruptComplete.ModbusGateway.4) OTL(@e392d01d@.Util.Block.InterruptPending.ModbusGateway.4) ,XIC(@e392d01d@.ModbusGateway.Command[5].Trigger) XIO(@e392d01d@.Util.Block.InterruptComplete.ModbusGateway.5) OTL(@e392d01d@.Util.Block.InterruptPending.ModbusGateway.5) ,XIC(@e392d01d@.ModbusGateway.Command[6].Trigger) XIO(@e392d01d@.Util.Block.InterruptComplete.ModbusGateway.6) OTL(@e392d01d@.Util.Block.InterruptPending.ModbusGateway.6) ,XIC(@e392d01d@.ModbusGateway.Command[7].Trigger) XIO(@e392d01d@.Util.Block.InterruptComplete.ModbusGateway.7) OTL(@e392d01d@.Util.Block.InterruptPending.ModbusGateway.7) ,XIC(@e392d01d@.ModbusGateway.Command[8].Trigger) XIO(@e392d01d@.Util.Block.InterruptComplete.ModbusGateway.8) OTL(@e392d01d@.Util.Block.InterruptPending.ModbusGateway.8) ,XIC(@e392d01d@.ModbusGateway.Command[9].Trigger) XIO(@e392d01d@.Util.Block.InterruptComplete.ModbusGateway.9) OTL(@e392d01d@.Util.Block.InterruptPending.ModbusGateway.9) ,XIC(@e392d01d@.Util.Block.InterruptPending.EnableDisable) XIO(@e392d01d@.Util.Block.InterruptComplete.EnableDisable) ,XIC(@e392d01d@.Util.Block.InterruptPending.Analysis.0) XIO(@e392d01d@.Util.Block.InterruptComplete.Analysis.0) ,XIC(@e392d01d@.Util.Block.InterruptPending.Analysis.1) XIO(@e392d01d@.Util.Block.InterruptComplete.Analysis.1) ,XIC(@e392d01d@.Util.Block.InterruptPending.Analysis.2) XIO(@e392d01d@.Util.Block.InterruptComplete.Analysis.2) ,XIC(@e392d01d@.Util.Block.InterruptPending.Analysis.3) XIO(@e392d01d@.Util.Block.InterruptComplete.Analysis.3) ,XIC(@e392d01d@.Util.Block.InterruptPending.Analysis.4) XIO(@e392d01d@.Util.Block.InterruptComplete.Analysis.4) ,XIC(@e392d01d@.Util.Block.InterruptPending.Analysis.5) XIO(@e392d01d@.Util.Block.InterruptComplete.Analysis.5) ]OTL(@e392d01d@.Util.Block.InterruptPending.Now);
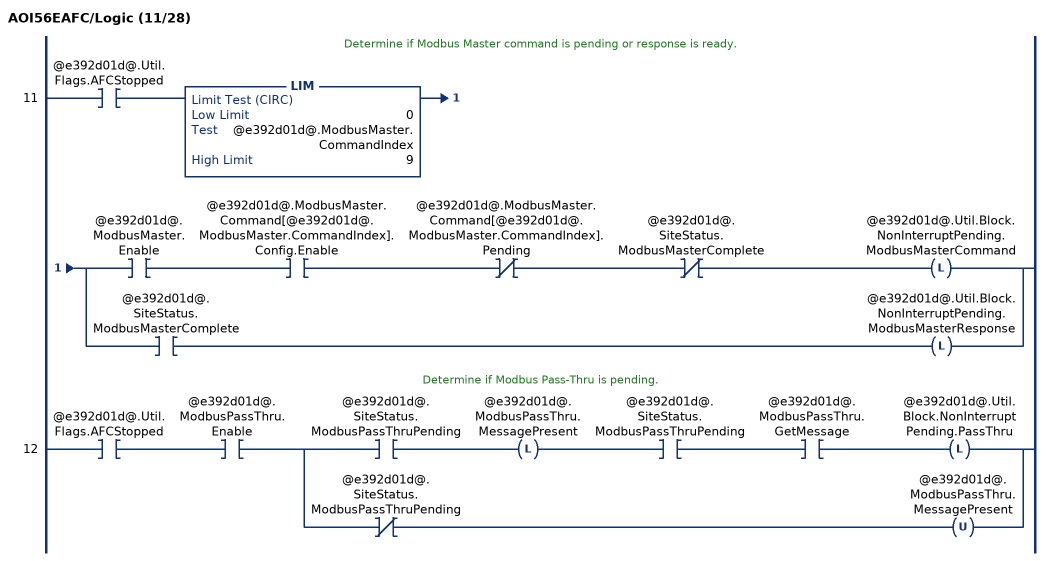
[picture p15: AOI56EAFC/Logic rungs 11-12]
   // Determine if Modbus Master command is pending or response is ready.
   11: XIC(@e392d01d@.Util.Flags.AFCStopped)LIM(0,@e392d01d@.ModbusMaster.CommandIndex,9)[XIC(@e392d01d@.ModbusMaster.Enable) XIC(@e392d01d@.ModbusMaster.Command[@e392d01d@.ModbusMaster.CommandIndex].Config.Enable) XIO(@e392d01d@.ModbusMaster.Command[@e392d01d@.ModbusMaster.CommandIndex].Pending) XIO(@e392d01d@.SiteStatus.ModbusMasterComplete) OTL(@e392d01d@.Util.Block.NonInterruptPending.ModbusMasterCommand) ,XIC(@e392d01d@.SiteStatus.ModbusMasterComplete) OTL(@e392d01d@.Util.Block.NonInterruptPending.ModbusMasterResponse) ];
   // Determine if Modbus Pass-Thru is pending.
   12: XIC(@e392d01d@.Util.Flags.AFCStopped)XIC(@e392d01d@.ModbusPassThru.Enable)[XIC(@e392d01d@.SiteStatus.ModbusPassThruPending) OTL(@e392d01d@.ModbusPassThru.MessagePresent) XIC(@e392d01d@.SiteStatus.ModbusPassThruPending) XIC(@e392d01d@.ModbusPassThru.GetMessage) OTL(@e392d01d@.Util.Block.NonInterruptPending.PassThru) ,XIO(@e392d01d@.SiteStatus.ModbusPassThruPending) OTU(@e392d01d@.ModbusPassThru.MessagePresent) ];
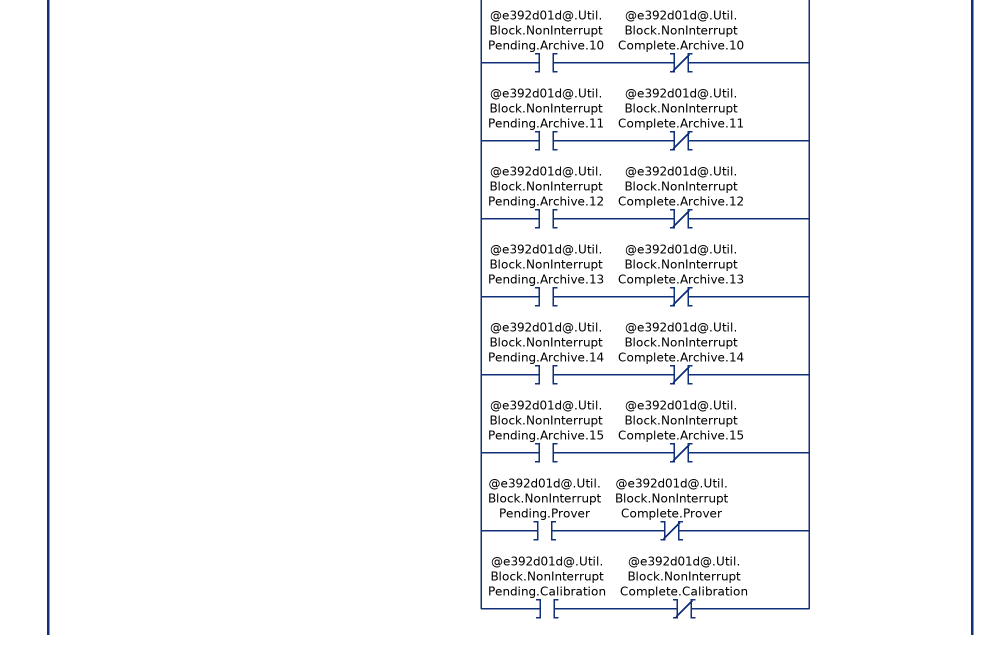
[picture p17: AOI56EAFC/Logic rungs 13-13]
   // Non-Interrupt blocks (1000, 2000 and 5000) occur after Process Input block 16.
   // Check if any non-interrupt block is pending.
   13: XIC(@e392d01d@.Util.Flags.AFCStopped)EQU(@e392d01d@.Util.Buffer.Input[0],16)[XIC(@e392d01d@.Util.Block.NonInterruptPending.ModbusMasterCommand) XIO(@e392d01d@.Util.Block.NonInterruptComplete.ModbusMasterCommand) ,XIC(@e392d01d@.Util.Block.NonInterruptPending.ModbusMasterResponse) XIO(@e392d01d@.Util.Block.NonInterruptComplete.ModbusMasterResponse) ,XIC(@e392d01d@.Util.Block.NonInterruptPending.PassThru) XIO(@e392d01d@.Util.Block.NonInterruptComplete.PassThru) ,XIC(@e392d01d@.Util.Block.NonInterruptPending.Archive.0) XIO(@e392d01d@.Util.Block.NonInterruptComplete.Archive.0) ,XIC(@e392d01d@.Util.Block.NonInterruptPending.Archive.1) XIO(@e392d01d@.Util.Block.NonInterruptComplete.Archive.1) ,XIC(@e392d01d@.Util.Block.NonInterruptPending.Archive.2) XIO(@e392d01d@.Util.Block.NonInterruptComplete.Archive.2) ,XIC(@e392d01d@.Util.Block.NonInterruptPending.Archive.3) XIO(@e392d01d@.Util.Block.NonInterruptComplete.Archive.3) ,XIC(@e392d01d@.Util.Block.NonInterruptPending.Archive.4) XIO(@e392d01d@.Util.Block.NonInterruptComplete.Archive.4) ,XIC(@e392d01d@.Util.Block.NonInterruptPending.Archive.5) XIO(@e392d01d@.Util.Block.NonInterruptComplete.Archive.5) ,XIC(@e392d01d@.Util.Block.NonInterruptPending.Archive.6) XIO(@e392d01d@.Util.Block.NonInterruptComplete.Archive.6) ,XIC(@e392d01d@.Util.Block.NonInterruptPending.Archive.7) XIO(@e392d01d@.Util.Block.NonInterruptComplete.Archive.7) ,XIC(@e392d01d@.Util.Block.NonInterruptPending.Archive.8) XIO(@e392d01d@.Util.Block.NonInterruptComplete.Archive.8) ,XIC(@e392d01d@.Util.Block.NonInterruptPending.Archive.9) XIO(@e392d01d@.Util.Block.NonInterruptComplete.Archive.9) ,XIC(@e392d01d@.Util.Block.NonInterruptPending.Archive.10) XIO(@e392d01d@.Util.Block.NonInterruptComplete.Archive.10) ,XIC(@e392d01d@.Util.Block.NonInterruptPending.Archive.11) XIO(@e392d01d@.Util.Block.NonInterruptComplete.Archive.11) ,XIC(@e392d01d@.Util.Block.NonInterruptPending.Archive.12) XIO(@e392d01d@.Util.Block.NonInterruptComplete.Archive.12) ,XIC(@e392d01d@.Util.Block.NonInterruptPending.Archive.13) XIO(@e392d01d@.Util.Block.NonInterruptComplete.Archive.13) ,XIC(@e392d01d@.Util.Block.NonInterruptPending.Archive.14) XIO(@e392d01d@.Util.Block.NonInterruptComplete.Archive.14) ,XIC(@e392d01d@.Util.Block.NonInterruptPending.Archive.15) XIO(@e392d01d@.Util.Block.NonInterruptComplete.Archive.15) ,XIC(@e392d01d@.Util.Block.NonInterruptPending.Prover) XIO(@e392d01d@.Util.Block.NonInterruptComplete.Prover) ,XIC(@e392d01d@.Util.Block.NonInterruptPending.Calibration) XIO(@e392d01d@.Util.Block.NonInterruptComplete.Calibration) ]OTL(@e392d01d@.Util.Block.NonInterruptPending.Now);
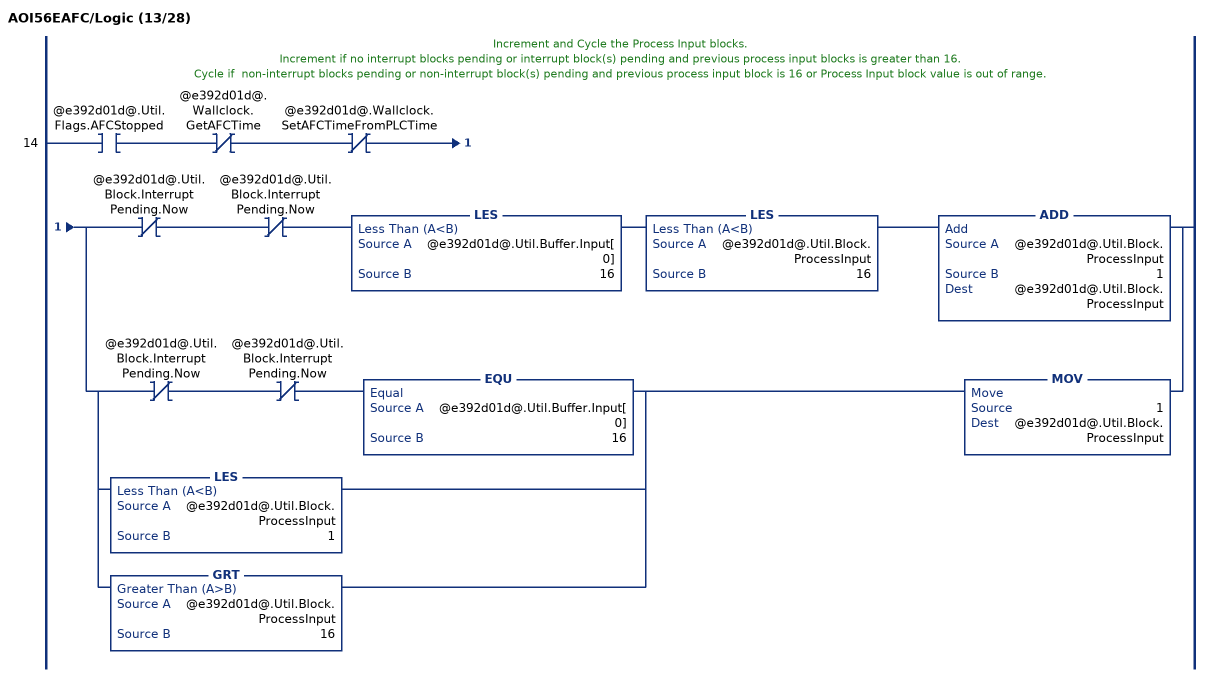
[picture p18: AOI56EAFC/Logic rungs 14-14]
   // Increment and Cycle the Process Input blocks.
   // Increment if no interrupt blocks pending or interrupt block(s) pending and previous process input blocks is greater than 16.
   // Cycle if  non-interrupt blocks pending or non-interrupt block(s) pending and previous process input block is 16 or Process Input block value is out of range.
   14: XIC(@e392d01d@.Util.Flags.AFCStopped)XIO(@e392d01d@.Wallclock.GetAFCTime)XIO(@e392d01d@.Wallclock.SetAFCTimeFromPLCTime)[XIO(@e392d01d@.Util.Block.InterruptPending.Now) XIO(@e392d01d@.Util.Block.InterruptPending.Now) LES(@e392d01d@.Util.Buffer.Input[0],16) LES(@e392d01d@.Util.Block.ProcessInput,16) ADD(@e392d01d@.Util.Block.ProcessInput,1,@e392d01d@.Util.Block.ProcessInput) ,[XIO(@e392d01d@.Util.Block.InterruptPending.Now) XIO(@e392d01d@.Util.Block.InterruptPending.Now) EQU(@e392d01d@.Util.Buffer.Input[0],16) ,LES(@e392d01d@.Util.Block.ProcessInput,1) ,GRT(@e392d01d@.Util.Block.ProcessInput,16) ] MOV(1,@e392d01d@.Util.Block.ProcessInput) ];
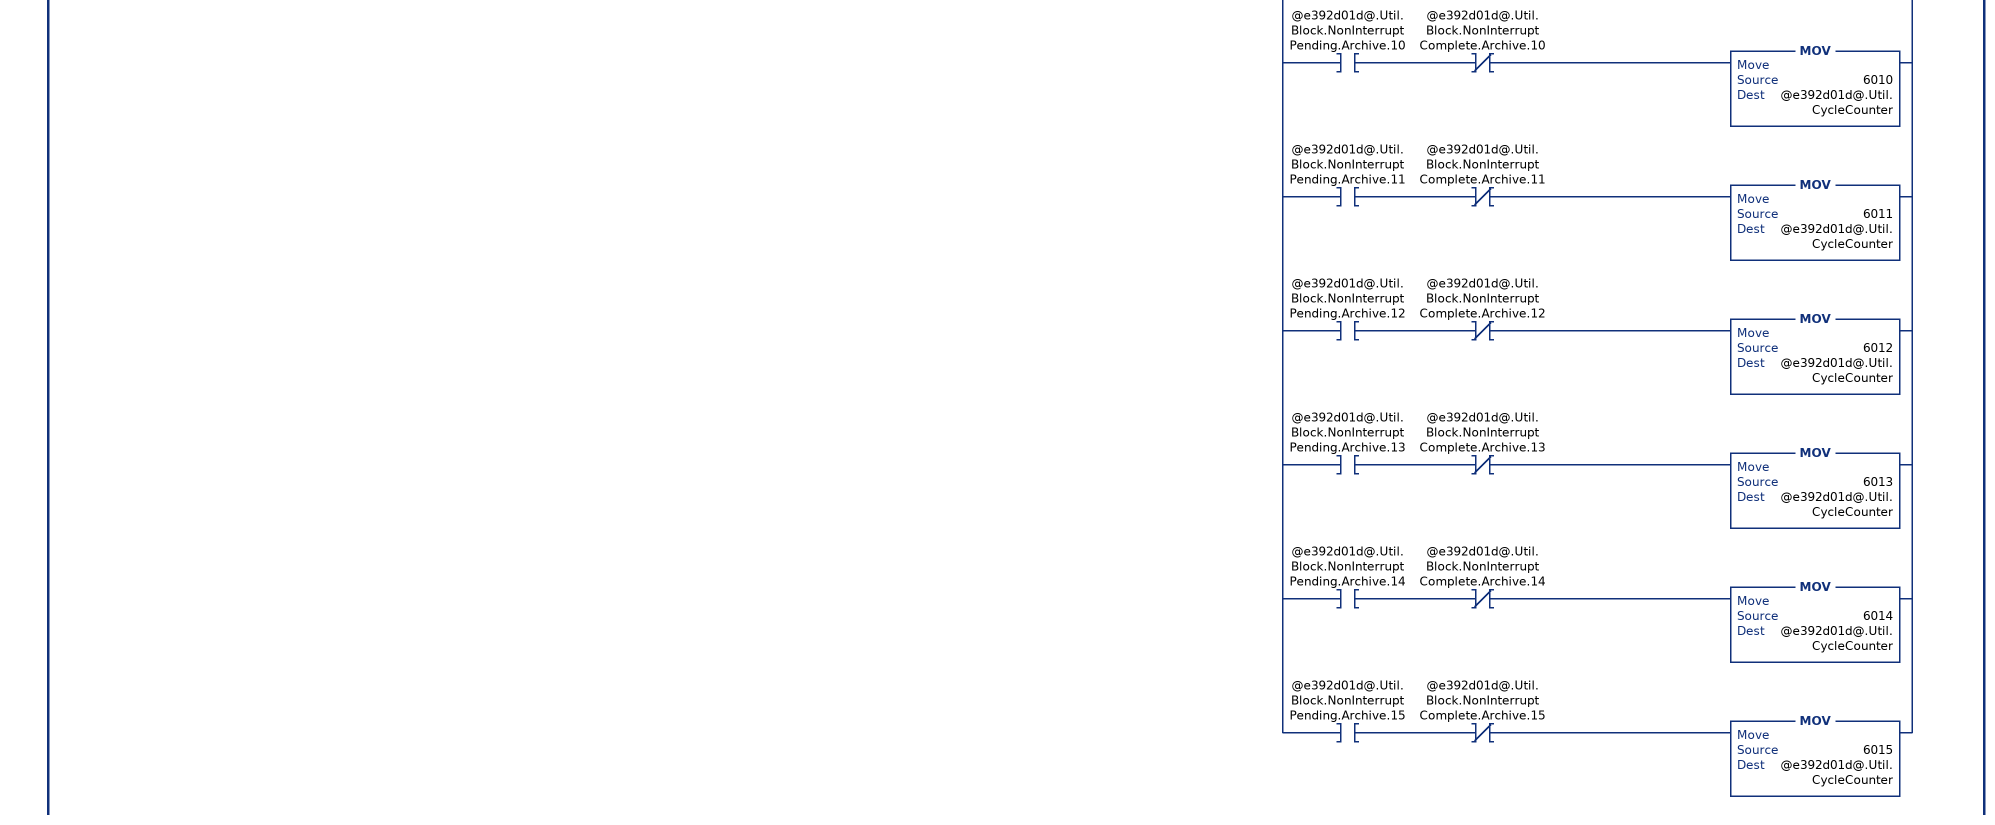
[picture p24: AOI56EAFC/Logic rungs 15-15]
   // Determine the next block to send to module.
   // Send Process Input block if previous block is interrupt or non-interrupt block or either block type is not pending.
   // Send Interrupt block if previous block is Process Input block 1-15 and interrupt block pending.
   // Send Non-interrupt block if previous block is Process Input block 16 and non-interrupt block pending.
   // Note: the block ID has no meaning to the AFC module. The module only requires that the ID changes.
   15: XIC(@e392d01d@.Util.Flags.AFCStopped)XIO(@e392d01d@.Wallclock.GetAFCTime)XIO(@e392d01d@.Wallclock.SetAFCTimeFromPLCTime)[[XIO(@e392d01d@.Util.Block.InterruptPending.Now) LIM(1,@e392d01d@.Util.Buffer.Input[0],15) ,XIO(@e392d01d@.Util.Block.NonInterruptPending.Now) EQU(@e392d01d@.Util.Buffer.Input[0],16) ,GRT(@e392d01d@.Util.Buffer.Input[0],16) ] MOV(@e392d01d@.Util.Block.ProcessInput,@e392d01d@.Util.CycleCounter) ,XIC(@e392d01d@.Util.Block.InterruptPending.Now) LIM(1,@e392d01d@.Util.Buffer.Input[0],15) [[XIC(@e392d01d@.Util.Block.InterruptPending.ModbusGateway.0) XIO(@e392d01d@.Util.Block.InterruptComplete.ModbusGateway.0) MOV(4000,@e392d01d@.Util.CycleCounter) ,XIC(@e392d01d@.Util.Block.InterruptPending.ModbusGateway.1) XIO(@e392d01d@.Util.Block.InterruptComplete.ModbusGateway.1) MOV(4001,@e392d01d@.Util.CycleCounter) ,XIC(@e392d01d@.Util.Block.InterruptPending.ModbusGateway.2) XIO(@e392d01d@.Util.Block.InterruptComplete.ModbusGateway.2) MOV(4002,@e392d01d@.Util.CycleCounter) ,XIC(@e392d01d@.Util.Block.InterruptPending.ModbusGateway.3) XIO(@e392d01d@.Util.Block.InterruptComplete.ModbusGateway.3) MOV(4003,@e392d01d@.Util.CycleCounter) ,XIC(@e392d01d@.Util.Block.InterruptPending.ModbusGateway.4) XIO(@e392d01d@.Util.Block.InterruptComplete.ModbusGateway.4) MOV(4004,@e392d01d@.Util.CycleCounter) ,XIC(@e392d01d@.Util.Block.InterruptPending.ModbusGateway.5) XIO(@e392d01d@.Util.Block.InterruptComplete.ModbusGateway.5) MOV(4005,@e392d01d@.Util.CycleCounter) ,XIC(@e392d01d@.Util.Block.InterruptPending.ModbusGateway.6) XIO(@e392d01d@.Util.Block.InterruptComplete.ModbusGateway.6) MOV(4006,@e392d01d@.Util.CycleCounter) ,XIC(@e392d01d@.Util.Block.InterruptPending.ModbusGateway.7) XIO(@e392d01d@.Util.Block.InterruptComplete.ModbusGateway.7) MOV(4007,@e392d01d@.Util.CycleCounter) ,XIC(@e392d01d@.Util.Block.InterruptPending.ModbusGateway.8) XIO(@e392d01d@.Util.Block.InterruptComplete.ModbusGateway.8) MOV(4008,@e392d01d@.Util.CycleCounter) ,XIC(@e392d01d@.Util.Block.InterruptPending.ModbusGateway.9) XIO(@e392d01d@.Util.Block.InterruptComplete.ModbusGateway.9) MOV(4009,@e392d01d@.Util.CycleCounter) ] ,EQU(@e392d01d@.Util.Block.InterruptPending.ModbusGateway,0) XIC(@e392d01d@.Util.Block.InterruptPending.EnableDisable) XIO(@e392d01d@.Util.Block.InterruptComplete.EnableDisable) MOV(7000,@e392d01d@.Util.CycleCounter) ,EQU(@e392d01d@.Util.Block.InterruptPending.ModbusGateway,0) XIO(@e392d01d@.Util.Block.InterruptPending.EnableDisable) [XIC(@e392d01d@.Util.Block.InterruptPending.Analysis.0) XIO(@e392d01d@.Util.Block.InterruptComplete.Analysis.0) MOV(3000,@e392d01d@.Util.CycleCounter) ,XIC(@e392d01d@.Util.Block.InterruptPending.Analysis.1) XIO(@e392d01d@.Util.Block.InterruptComplete.Analysis.1) MOV(3001,@e392d01d@.Util.CycleCounter) ,XIC(@e392d01d@.Util.Block.InterruptPending.Analysis.2) XIO(@e392d01d@.Util.Block.InterruptComplete.Analysis.2) MOV(3002,@e392d01d@.Util.CycleCounter) ,XIC(@e392d01d@.Util.Block.InterruptPending.Analysis.3) XIO(@e392d01d@.Util.Block.InterruptComplete.Analysis.3) MOV(3003,@e392d01d@.Util.CycleCounter) ,XIC(@e392d01d@.Util.Block.InterruptPending.Analysis.4) XIO(@e392d01d@.Util.Block.InterruptComplete.Analysis.4) MOV(3004,@e392d01d@.Util.CycleCounter) ,XIC(@e392d01d@.Util.Block.InterruptPending.Analysis.5) XIO(@e392d01d@.Util.Block.InterruptComplete.Analysis.5) MOV(3005,@e392d01d@.Util.CycleCounter) ] ] ,XIC(@e392d01d@.Util.Block.NonInterruptPending.Now) EQU(@e392d01d@.Util.Buffer.Input[0],16) [XIC(@e392d01d@.ModbusMaster.Enable) LIM(0,@e392d01d@.ModbusMaster.CommandIndex,9) [XIO(@e392d01d@.Util.Block.NonInterruptComplete.ModbusMasterCommand) XIC(@e392d01d@.ModbusMaster.Command[@e392d01d@.ModbusMaster.CommandIndex].Config.Enable) XIO(@e392d01d@.SiteStatus.ModbusMasterPending) XIO(@e392d01d@.SiteStatus.ModbusMasterComplete) MOV(1000,@e392d01d@.Util.CycleCounter) ,XIO(@e392d01d@.Util.Block.NonInterruptComplete.ModbusMasterResponse) XIC(@e392d01d@.SiteStatus.ModbusMasterComplete) MOV(1001,@e392d01d@.Util.CycleCounter) ] ,XIO(@e392d01d@.Util.Block.NonInterruptPending.ModbusMasterCommand) XIO(@e392d01d@.Util.Block.NonInterruptPending.ModbusMasterResponse) [XIC(@e392d01d@.ModbusPassThru.Enable) XIC(@e392d01d@.SiteStatus.ModbusPassThruPending) XIC(@e392d01d@.ModbusPassThru.GetMessage) MOV(2000,@e392d01d@.Util.CycleCounter) ,XIO(@e392d01d@.Util.Block.NonInterruptPending.PassThru) [XIC(@e392d01d@.Util.Block.NonInterruptPending.Prover) XIO(@e392d01d@.Util.Block.NonInterruptComplete.Prover) XIC(@e392d01d@.Prove.ProveEnabled) MOV(5000,@e392d01d@.Util.CycleCounter) ,XIO(@e392d01d@.Util.Block.NonInterruptPending.Prover) [XIC(@e392d01d@.SiteStatus.CalibrationRequest) XIO(@e392d01d@.Util.Block.NonInterruptComplete.Calibration) [EQU(@e392d01d@.Util.Buffer.Calibration[1],0) MOV(9000,@e392d01d@.Util.CycleCounter) ,NEQ(@e392d01d@.Util.Buffer.Calibration[1],0) MOV(9001,@e392d01d@.Util.CycleCounter) ] ,XIO(@e392d01d@.Util.Block.NonInterruptPending.Calibration) [XIC(@e392d01d@.Util.Block.NonInterruptPending.Archive.0) XIO(@e392d01d@.Util.Block.NonInterruptComplete.Archive.0) MOV(6000,@e392d01d@.Util.CycleCounter) ,XIC(@e392d01d@.Util.Block.NonInterruptPending.Archive.1) XIO(@e392d01d@.Util.Block.NonInterruptComplete.Archive.1) MOV(6001,@e392d01d@.Util.CycleCounter) ,XIC(@e392d01d@.Util.Block.NonInterruptPending.Archive.2) XIO(@e392d01d@.Util.Block.NonInterruptComplete.Archive.2) MOV(6002,@e392d01d@.Util.CycleCounter) ,XIC(@e392d01d@.Util.Block.NonInterruptPending.Archive.3) XIO(@e392d01d@.Util.Block.NonInterruptComplete.Archive.3) MOV(6003,@e392d01d@.Util.CycleCounter) ,XIC(@e392d01d@.Util.Block.NonInterruptPending.Archive.4) XIO(@e392d01d@.Util.Block.NonInterruptComplete.Archive.4) MOV(6004,@e392d01d@.Util.CycleCounter) ,XIC(@e392d01d@.Util.Block.NonInterruptPending.Archive.5) XIO(@e392d01d@.Util.Block.NonInterruptComplete.Archive.5) MOV(6005,@e392d01d@.Util.CycleCounter) ,XIC(@e392d01d@.Util.Block.NonInterruptPending.Archive.6) XIO(@e392d01d@.Util.Block.NonInterruptComplete.Archive.6) MOV(6006,@e392d01d@.Util.CycleCounter) ,XIC(@e392d01d@.Util.Block.NonInterruptPending.Archive.7) XIO(@e392d01d@.Util.Block.NonInterruptComplete.Archive.7) MOV(6007,@e392d01d@.Util.CycleCounter) ,XIC(@e392d01d@.Util.Block.NonInterruptPending.Archive.8) XIO(@e392d01d@.Util.Block.NonInterruptComplete.Archive.8) MOV(6008,@e392d01d@.Util.CycleCounter) ,XIC(@e392d01d@.Util.Block.NonInterruptPending.Archive.9) XIO(@e392d01d@.Util.Block.NonInterruptComplete.Archive.9) MOV(6009,@e392d01d@.Util.CycleCounter) ,XIC(@e392d01d@.Util.Block.NonInterruptPending.Archive.10) XIO(@e392d01d@.Util.Block.NonInterruptComplete.Archive.10) MOV(6010,@e392d01d@.Util.CycleCounter) ,XIC(@e392d01d@.Util.Block.NonInterruptPending.Archive.11) XIO(@e392d01d@.Util.Block.NonInterruptComplete.Archive.11) MOV(6011,@e392d01d@.Util.CycleCounter) ,XIC(@e392d01d@.Util.Block.NonInterruptPending.Archive.12) XIO(@e392d01d@.Util.Block.NonInterruptComplete.Archive.12) MOV(6012,@e392d01d@.Util.CycleCounter) ,XIC(@e392d01d@.Util.Block.NonInterruptPending.Archive.13) XIO(@e392d01d@.Util.Block.NonInterruptComplete.Archive.13) MOV(6013,@e392d01d@.Util.CycleCounter) ,XIC(@e392d01d@.Util.Block.NonInterruptPending.Archive.14) XIO(@e392d01d@.Util.Block.NonInterruptComplete.Archive.14) MOV(6014,@e392d01d@.Util.CycleCounter) ,XIC(@e392d01d@.Util.Block.NonInterruptPending.Archive.15) XIO(@e392d01d@.Util.Block.NonInterruptComplete.Archive.15) MOV(6015,@e392d01d@.Util.CycleCounter) ] ] ] ] ] ];
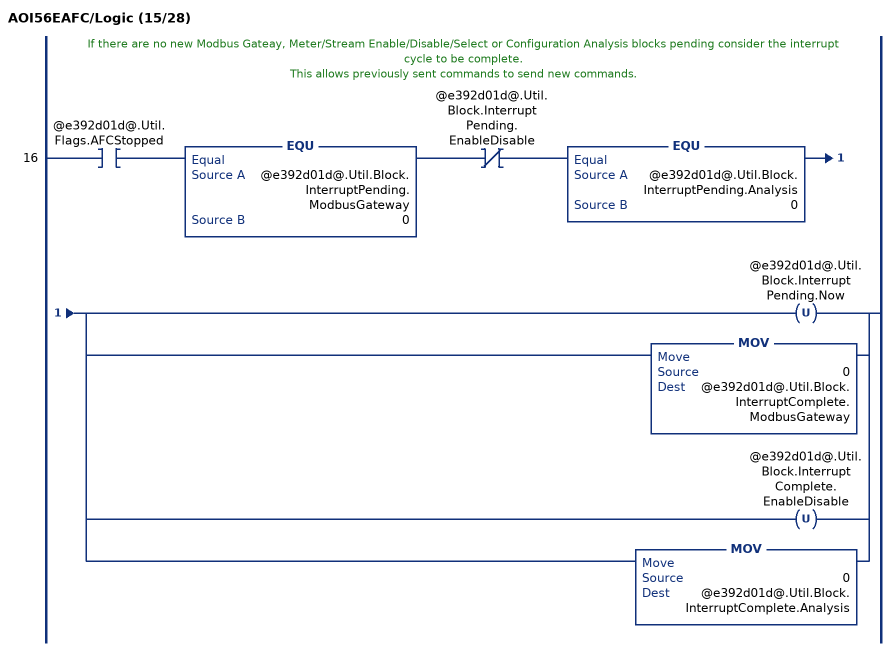
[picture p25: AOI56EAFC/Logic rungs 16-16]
   // If there are no new Modbus Gateay, Meter/Stream Enable/Disable/Select or Configuration Analysis blocks pending consider the interrupt cycle to be complete.
   // This allows previously sent commands to send new commands.
   16: XIC(@e392d01d@.Util.Flags.AFCStopped)EQU(@e392d01d@.Util.Block.InterruptPending.ModbusGateway,0)XIO(@e392d01d@.Util.Block.InterruptPending.EnableDisable)EQU(@e392d01d@.Util.Block.InterruptPending.Analysis,0)[OTU(@e392d01d@.Util.Block.InterruptPending.Now) ,MOV(0,@e392d01d@.Util.Block.InterruptComplete.ModbusGateway) ,OTU(@e392d01d@.Util.Block.InterruptComplete.EnableDisable) ,MOV(0,@e392d01d@.Util.Block.InterruptComplete.Analysis) ];
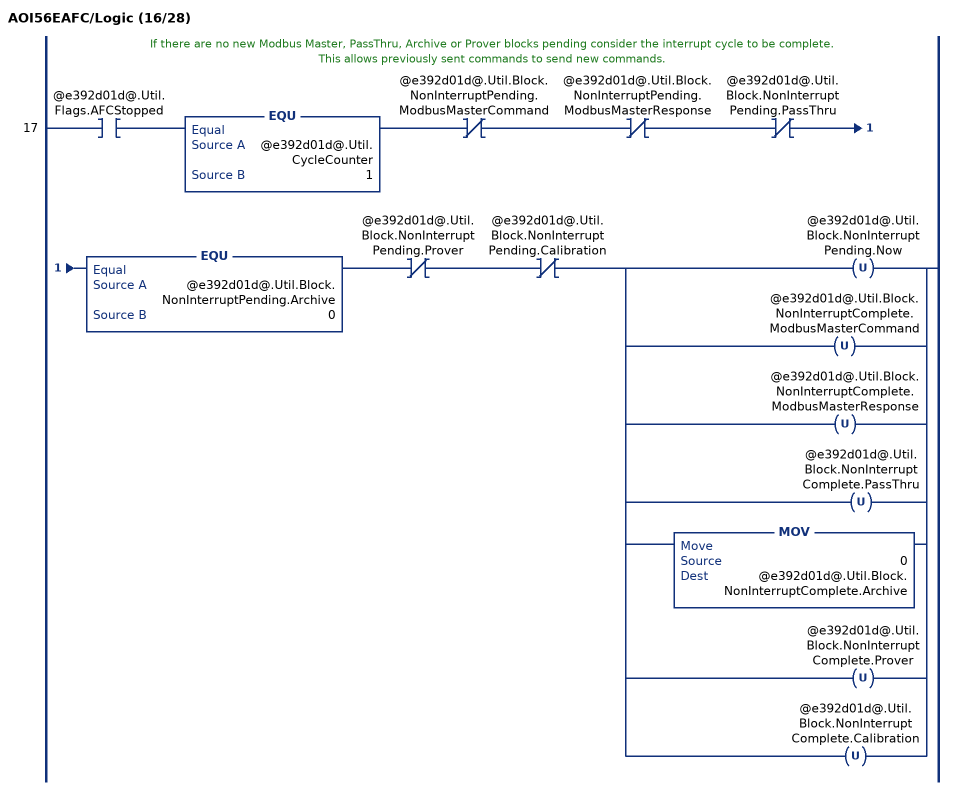
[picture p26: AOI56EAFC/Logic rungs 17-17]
   // If there are no new Modbus Master, PassThru, Archive or Prover blocks pending consider the interrupt cycle to be complete.
   // This allows previously sent commands to send new commands.
   17: XIC(@e392d01d@.Util.Flags.AFCStopped)EQU(@e392d01d@.Util.CycleCounter,1)XIO(@e392d01d@.Util.Block.NonInterruptPending.ModbusMasterCommand)XIO(@e392d01d@.Util.Block.NonInterruptPending.ModbusMasterResponse)XIO(@e392d01d@.Util.Block.NonInterruptPending.PassThru)EQU(@e392d01d@.Util.Block.NonInterruptPending.Archive,0)XIO(@e392d01d@.Util.Block.NonInterruptPending.Prover)XIO(@e392d01d@.Util.Block.NonInterruptPending.Calibration)[OTU(@e392d01d@.Util.Block.NonInterruptPending.Now) ,OTU(@e392d01d@.Util.Block.NonInterruptComplete.ModbusMasterCommand) ,OTU(@e392d01d@.Util.Block.NonInterruptComplete.ModbusMasterResponse) ,OTU(@e392d01d@.Util.Block.NonInterruptComplete.PassThru) ,MOV(0,@e392d01d@.Util.Block.NonInterruptComplete.Archive) ,OTU(@e392d01d@.Util.Block.NonInterruptComplete.Prover) ,OTU(@e392d01d@.Util.Block.NonInterruptComplete.Calibration) ];
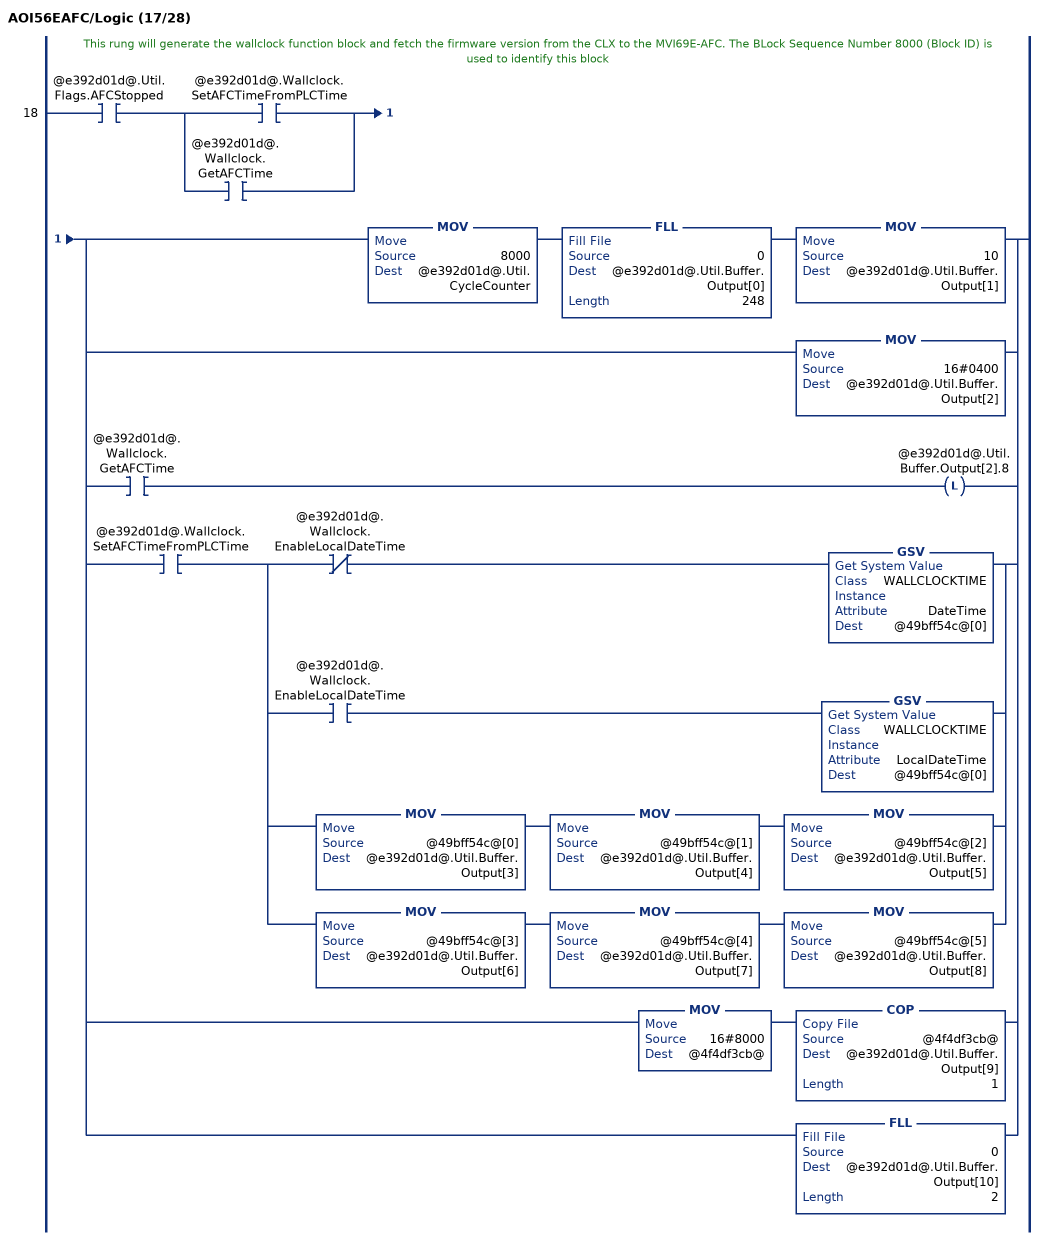
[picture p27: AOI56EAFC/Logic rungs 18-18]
   // This rung will generate the wallclock function block and fetch the firmware version from the CLX to the MVI69E-AFC. The BLock Sequence Number 8000 (Block ID) is used to identify this block
   18: XIC(@e392d01d@.Util.Flags.AFCStopped)[XIC(@e392d01d@.Wallclock.SetAFCTimeFromPLCTime) ,XIC(@e392d01d@.Wallclock.GetAFCTime) ][MOV(8000,@e392d01d@.Util.CycleCounter) FLL(0,@e392d01d@.Util.Buffer.Output[0],248) MOV(10,@e392d01d@.Util.Buffer.Output[1]) ,[MOV(16#0400,@e392d01d@.Util.Buffer.Output[2]) ,XIC(@e392d01d@.Wallclock.GetAFCTime) OTL(@e392d01d@.Util.Buffer.Output[2].8) ] ,XIC(@e392d01d@.Wallclock.SetAFCTimeFromPLCTime) [[XIO(@e392d01d@.Wallclock.EnableLocalDateTime) GSV(WALLCLOCKTIME,,DateTime,@49bff54c@[0]) ,XIC(@e392d01d@.Wallclock.EnableLocalDateTime) GSV(WALLCLOCKTIME,,LocalDateTime,@49bff54c@[0]) ] ,MOV(@49bff54c@[0],@e392d01d@.Util.Buffer.Output[3]) MOV(@49bff54c@[1],@e392d01d@.Util.Buffer.Output[4]) MOV(@49bff54c@[2],@e392d01d@.Util.Buffer.Output[5]) ,MOV(@49bff54c@[3],@e392d01d@.Util.Buffer.Output[6]) MOV(@49bff54c@[4],@e392d01d@.Util.Buffer.Output[7]) MOV(@49bff54c@[5],@e392d01d@.Util.Buffer.Output[8]) ] ,[MOV(16#8000,@4f4df3cb@) COP(@4f4df3cb@,@e392d01d@.Util.Buffer.Output[9],1) ,FLL(0,@e392d01d@.Util.Buffer.Output[10],2) ] ];
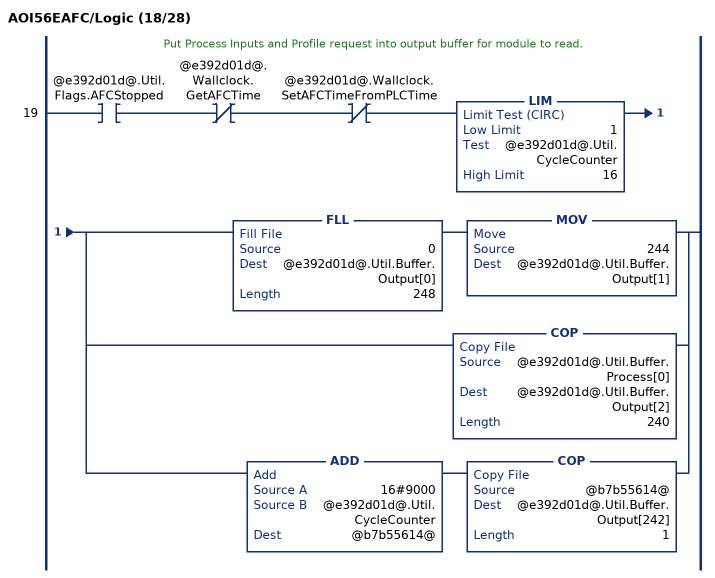
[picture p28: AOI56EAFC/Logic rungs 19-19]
   // Put Process Inputs and Profile request into output buffer for module to read.
   19: XIC(@e392d01d@.Util.Flags.AFCStopped)XIO(@e392d01d@.Wallclock.GetAFCTime)XIO(@e392d01d@.Wallclock.SetAFCTimeFromPLCTime)LIM(1,@e392d01d@.Util.CycleCounter,16)[FLL(0,@e392d01d@.Util.Buffer.Output[0],248) MOV(244,@e392d01d@.Util.Buffer.Output[1]) ,COP(@e392d01d@.Util.Buffer.Process[0],@e392d01d@.Util.Buffer.Output[2],240) ,ADD(16#9000,@e392d01d@.Util.CycleCounter,@b7b55614@) COP(@b7b55614@,@e392d01d@.Util.Buffer.Output[242],1) ];
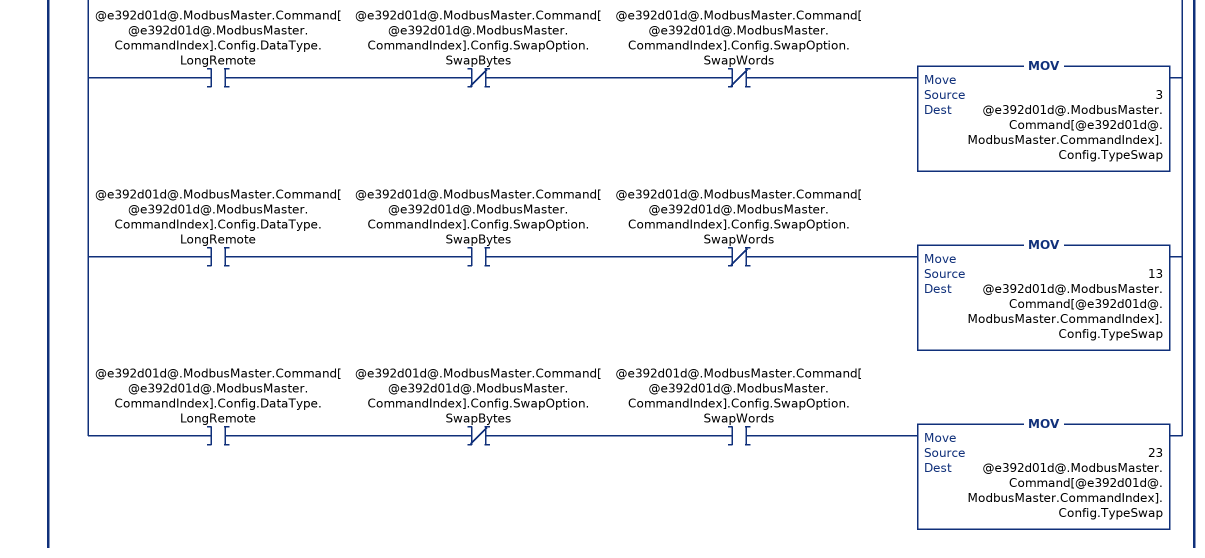
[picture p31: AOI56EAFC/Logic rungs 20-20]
   // Setup Modbus Master command.
   20: XIC(@e392d01d@.Util.Flags.AFCStopped)XIO(@e392d01d@.Wallclock.GetAFCTime)XIO(@e392d01d@.Wallclock.SetAFCTimeFromPLCTime)XIC(@e392d01d@.ModbusMaster.Enable)LIM(0,@e392d01d@.ModbusMaster.CommandIndex,9)[EQU(@e392d01d@.Util.CycleCounter,1000) XIO(@e392d01d@.Util.Block.NonInterruptComplete.ModbusMasterCommand) ,EQU(@e392d01d@.Util.CycleCounter,1001) XIO(@e392d01d@.Util.Block.NonInterruptComplete.ModbusMasterResponse) ][ADD(16#6000,130,@2d1a8896@) ,[XIC(@e392d01d@.ModbusMaster.Command[@e392d01d@.ModbusMaster.CommandIndex].Config.FunctionType) [OTE(@2d1a8896@.11) ,OTL(@d09c43dc@) ] ,XIO(@e392d01d@.ModbusMaster.Command[@e392d01d@.ModbusMaster.CommandIndex].Config.FunctionType) OTU(@d09c43dc@) ] ,XIO(@e392d01d@.ModbusMaster.Command[@e392d01d@.ModbusMaster.CommandIndex].Config.Enable) OTE(@2d1a8896@.8) ,XIC(@e392d01d@.ModbusMaster.Command[@e392d01d@.ModbusMaster.CommandIndex].Config.RegisterBank) OTE(@2d1a8896@.10) ,XIC(@e392d01d@.ModbusMaster.Command[@e392d01d@.ModbusMaster.CommandIndex].Config.DataType.Bit) MOV(0,@e392d01d@.ModbusMaster.Command[@e392d01d@.ModbusMaster.CommandIndex].Config.TypeSwap) ,XIC(@e392d01d@.ModbusMaster.Command[@e392d01d@.ModbusMaster.CommandIndex].Config.DataType.Word) XIO(@e392d01d@.ModbusMaster.Command[@e392d01d@.ModbusMaster.CommandIndex].Config.SwapOption.SwapBytes) MOV(1,@e392d01d@.ModbusMaster.Command[@e392d01d@.ModbusMaster.CommandIndex].Config.TypeSwap) ,XIC(@e392d01d@.ModbusMaster.Command[@e392d01d@.ModbusMaster.CommandIndex].Config.DataType.Word) XIC(@e392d01d@.ModbusMaster.Command[@e392d01d@.ModbusMaster.CommandIndex].Config.SwapOption.SwapBytes) MOV(11,@e392d01d@.ModbusMaster.Command[@e392d01d@.ModbusMaster.CommandIndex].Config.TypeSwap) ,XIC(@e392d01d@.ModbusMaster.Command[@e392d01d@.ModbusMaster.CommandIndex].Config.DataType.Long) XIO(@e392d01d@.ModbusMaster.Command[@e392d01d@.ModbusMaster.CommandIndex].Config.SwapOption.SwapBytes) XIO(@e392d01d@.ModbusMaster.Command[@e392d01d@.ModbusMaster.CommandIndex].Config.SwapOption.SwapWords) MOV(2,@e392d01d@.ModbusMaster.Command[@e392d01d@.ModbusMaster.CommandIndex].Config.TypeSwap) ,XIC(@e392d01d@.ModbusMaster.Command[@e392d01d@.ModbusMaster.CommandIndex].Config.DataType.Long) XIC(@e392d01d@.ModbusMaster.Command[@e392d01d@.ModbusMaster.CommandIndex].Config.SwapOption.SwapBytes) XIO(@e392d01d@.ModbusMaster.Command[@e392d01d@.ModbusMaster.CommandIndex].Config.SwapOption.SwapWords) MOV(12,@e392d01d@.ModbusMaster.Command[@e392d01d@.ModbusMaster.CommandIndex].Config.TypeSwap) ,XIC(@e392d01d@.ModbusMaster.Command[@e392d01d@.ModbusMaster.CommandIndex].Config.DataType.Long) XIO(@e392d01d@.ModbusMaster.Command[@e392d01d@.ModbusMaster.CommandIndex].Config.SwapOption.SwapBytes) XIC(@e392d01d@.ModbusMaster.Command[@e392d01d@.ModbusMaster.CommandIndex].Config.SwapOption.SwapWords) MOV(22,@e392d01d@.ModbusMaster.Command[@e392d01d@.ModbusMaster.CommandIndex].Config.TypeSwap) ,XIC(@e392d01d@.ModbusMaster.Command[@e392d01d@.ModbusMaster.CommandIndex].Config.DataType.LongRemote) XIO(@e392d01d@.ModbusMaster.Command[@e392d01d@.ModbusMaster.CommandIndex].Config.SwapOption.SwapBytes) XIO(@e392d01d@.ModbusMaster.Command[@e392d01d@.ModbusMaster.CommandIndex].Config.SwapOption.SwapWords) MOV(3,@e392d01d@.ModbusMaster.Command[@e392d01d@.ModbusMaster.CommandIndex].Config.TypeSwap) ,XIC(@e392d01d@.ModbusMaster.Command[@e392d01d@.ModbusMaster.CommandIndex].Config.DataType.LongRemote) XIC(@e392d01d@.ModbusMaster.Command[@e392d01d@.ModbusMaster.CommandIndex].Config.SwapOption.SwapBytes) XIO(@e392d01d@.ModbusMaster.Command[@e392d01d@.ModbusMaster.CommandIndex].Config.SwapOption.SwapWords) MOV(13,@e392d01d@.ModbusMaster.Command[@e392d01d@.ModbusMaster.CommandIndex].Config.TypeSwap) ,XIC(@e392d01d@.ModbusMaster.Command[@e392d01d@.ModbusMaster.CommandIndex].Config.DataType.LongRemote) XIO(@e392d01d@.ModbusMaster.Command[@e392d01d@.ModbusMaster.CommandIndex].Config.SwapOption.SwapBytes) XIC(@e392d01d@.ModbusMaster.Command[@e392d01d@.ModbusMaster.CommandIndex].Config.SwapOption.SwapWords) MOV(23,@e392d01d@.ModbusMaster.Command[@e392d01d@.ModbusMaster.CommandIndex].Config.TypeSwap) ];
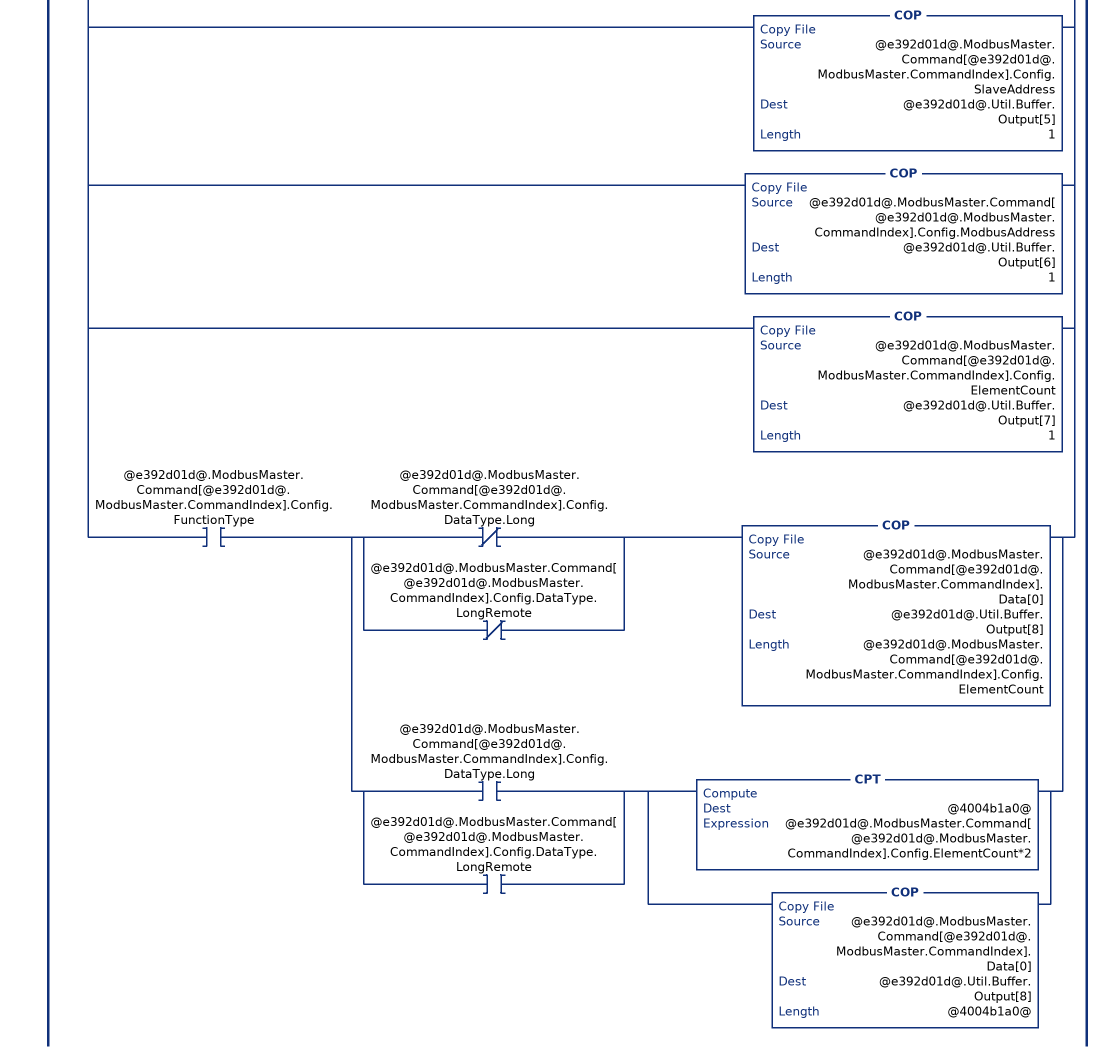
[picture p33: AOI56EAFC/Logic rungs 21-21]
   // Put Modbus Master command into output buffer for module to read.
   21: XIC(@e392d01d@.Util.Flags.AFCStopped)XIO(@e392d01d@.Wallclock.GetAFCTime)XIO(@e392d01d@.Wallclock.SetAFCTimeFromPLCTime)XIC(@e392d01d@.ModbusMaster.Enable)LIM(0,@e392d01d@.ModbusMaster.CommandIndex,9)[EQU(@e392d01d@.Util.CycleCounter,1000) XIO(@e392d01d@.Util.Block.NonInterruptComplete.ModbusMasterCommand) ,EQU(@e392d01d@.Util.CycleCounter,1001) XIO(@e392d01d@.Util.Block.NonInterruptComplete.ModbusMasterResponse) ][MOV(131,@e392d01d@.Util.Buffer.Output[1]) ,COP(@2d1a8896@,@e392d01d@.Util.Buffer.Output[2],1) ,COP(@e392d01d@.ModbusMaster.Command[@e392d01d@.ModbusMaster.CommandIndex].Config.TransactionID,@e392d01d@.Util.Buffer.Output[3],1) ,COP(@e392d01d@.ModbusMaster.Command[@e392d01d@.ModbusMaster.CommandIndex].Config.TypeSwap,@e392d01d@.Util.Buffer.Output[4],1) ,COP(@e392d01d@.ModbusMaster.Command[@e392d01d@.ModbusMaster.CommandIndex].Config.SlaveAddress,@e392d01d@.Util.Buffer.Output[5],1) ,COP(@e392d01d@.ModbusMaster.Command[@e392d01d@.ModbusMaster.CommandIndex].Config.ModbusAddress,@e392d01d@.Util.Buffer.Output[6],1) ,COP(@e392d01d@.ModbusMaster.Command[@e392d01d@.ModbusMaster.CommandIndex].Config.ElementCount,@e392d01d@.Util.Buffer.Output[7],1) ,XIC(@e392d01d@.ModbusMaster.Command[@e392d01d@.ModbusMaster.CommandIndex].Config.FunctionType) [[XIO(@e392d01d@.ModbusMaster.Command[@e392d01d@.ModbusMaster.CommandIndex].Config.DataType.Long) ,XIO(@e392d01d@.ModbusMaster.Command[@e392d01d@.ModbusMaster.CommandIndex].Config.DataType.LongRemote) ] COP(@e392d01d@.ModbusMaster.Command[@e392d01d@.ModbusMaster.CommandIndex].Data[0],@e392d01d@.Util.Buffer.Output[8],@e392d01d@.ModbusMaster.Command[@e392d01d@.ModbusMaster.CommandIndex].Config.ElementCount) ,[XIC(@e392d01d@.ModbusMaster.Command[@e392d01d@.ModbusMaster.CommandIndex].Config.DataType.Long) ,XIC(@e392d01d@.ModbusMaster.Command[@e392d01d@.ModbusMaster.CommandIndex].Config.DataType.LongRemote) ] [CPT(@4004b1a0@,@e392d01d@.ModbusMaster.Command[@e392d01d@.ModbusMaster.CommandIndex].Config.ElementCount*2) ,COP(@e392d01d@.ModbusMaster.Command[@e392d01d@.ModbusMaster.CommandIndex].Data[0],@e392d01d@.Util.Buffer.Output[8],@4004b1a0@) ] ] ];
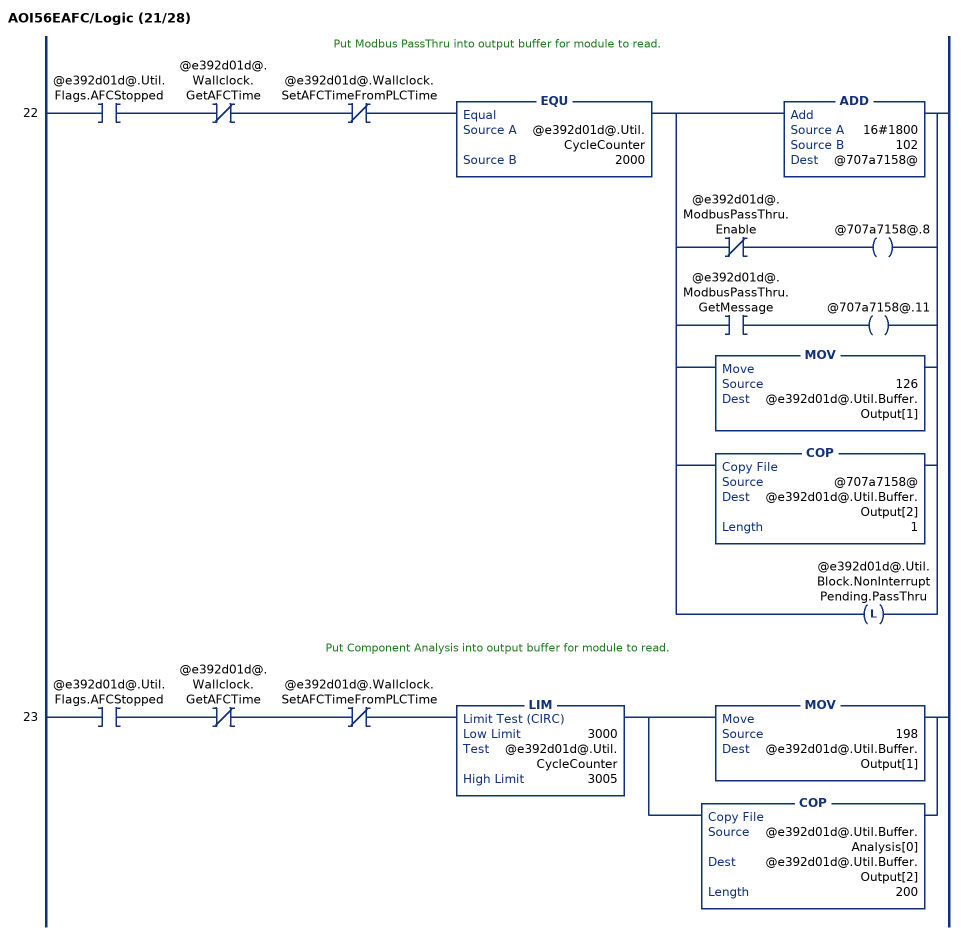
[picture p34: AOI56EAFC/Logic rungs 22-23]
   // Put Modbus PassThru into output buffer for module to read.
   22: XIC(@e392d01d@.Util.Flags.AFCStopped)XIO(@e392d01d@.Wallclock.GetAFCTime)XIO(@e392d01d@.Wallclock.SetAFCTimeFromPLCTime)EQU(@e392d01d@.Util.CycleCounter,2000)[ADD(16#1800,102,@707a7158@) ,XIO(@e392d01d@.ModbusPassThru.Enable) OTE(@707a7158@.8) ,XIC(@e392d01d@.ModbusPassThru.GetMessage) OTE(@707a7158@.11) ,MOV(126,@e392d01d@.Util.Buffer.Output[1]) ,COP(@707a7158@,@e392d01d@.Util.Buffer.Output[2],1) ,OTL(@e392d01d@.Util.Block.NonInterruptPending.PassThru) ];
   // Put Component Analysis into output buffer for module to read.
   23: XIC(@e392d01d@.Util.Flags.AFCStopped)XIO(@e392d01d@.Wallclock.GetAFCTime)XIO(@e392d01d@.Wallclock.SetAFCTimeFromPLCTime)LIM(3000,@e392d01d@.Util.CycleCounter,3005)[MOV(198,@e392d01d@.Util.Buffer.Output[1]) ,COP(@e392d01d@.Util.Buffer.Analysis[0],@e392d01d@.Util.Buffer.Output[2],200) ];
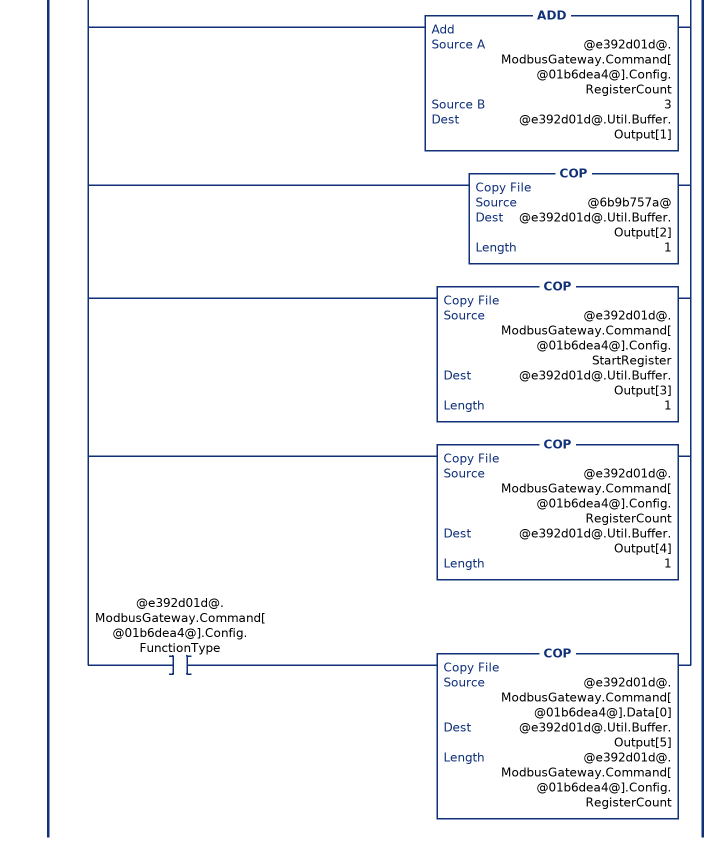
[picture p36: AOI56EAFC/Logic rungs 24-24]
   // Put Modbus Gateway command into output buffer for module to read.
   24: XIC(@e392d01d@.Util.Flags.AFCStopped)XIO(@e392d01d@.Wallclock.GetAFCTime)XIO(@e392d01d@.Wallclock.SetAFCTimeFromPLCTime)LIM(4000,@e392d01d@.Util.CycleCounter,4009)[SUB(@e392d01d@.Util.CycleCounter,4000,@01b6dea4@) CPT(@f96ca355@,2**@01b6dea4@) ,MOV(16#4000,@6b9b757a@) ,XIO(@e392d01d@.ModbusGateway.Command[@01b6dea4@].Config.Enable) OTE(@6b9b757a@.8) ,XIC(@e392d01d@.ModbusGateway.Command[@01b6dea4@].Config.SlaveType) OTE(@6b9b757a@.10) ,XIC(@e392d01d@.ModbusGateway.Command[@01b6dea4@].Config.RegisterType) OTE(@6b9b757a@.11) ,XIC(@e392d01d@.ModbusGateway.Command[@01b6dea4@].Config.FunctionType) OTE(@6b9b757a@.12) ,CPT(@6b9b757a@,@6b9b757a@+@e392d01d@.ModbusGateway.Command[@01b6dea4@].Config.RegisterCount+2) ,FLL(0,@e392d01d@.Util.Buffer.Output[1],246) ,ADD(@e392d01d@.ModbusGateway.Command[@01b6dea4@].Config.RegisterCount,3,@e392d01d@.Util.Buffer.Output[1]) ,COP(@6b9b757a@,@e392d01d@.Util.Buffer.Output[2],1) ,COP(@e392d01d@.ModbusGateway.Command[@01b6dea4@].Config.StartRegister,@e392d01d@.Util.Buffer.Output[3],1) ,COP(@e392d01d@.ModbusGateway.Command[@01b6dea4@].Config.RegisterCount,@e392d01d@.Util.Buffer.Output[4],1) ,XIC(@e392d01d@.ModbusGateway.Command[@01b6dea4@].Config.FunctionType) COP(@e392d01d@.ModbusGateway.Command[@01b6dea4@].Data[0],@e392d01d@.Util.Buffer.Output[5],@e392d01d@.ModbusGateway.Command[@01b6dea4@].Config.RegisterCount) ];
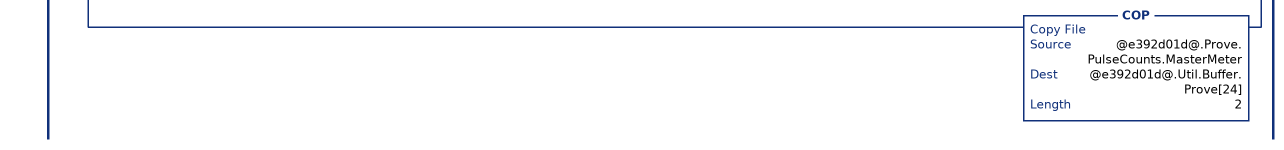
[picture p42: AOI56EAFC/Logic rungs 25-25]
   // The reason to check NEQ outputbuffer[0] 5000 is to guarantee the routine will be updated one time only, so the signals can be cleared correctly once the input block is received
   25: XIC(@e392d01d@.Prove.ProveEnabled)[NEQ(@e392d01d@.Util.Buffer.Output[0],5000) ,OTL(@e392d01d@.Util.Block.NonInterruptPending.Prover) ]EQU(@e392d01d@.Util.CycleCounter,5000)[MOV(0,@c3e12f53@) ,XIC(@e392d01d@.Prove.Process.Sequencing.Phase.NotSelected) [OTU(@c3e12f53@.0) ,OTU(@c3e12f53@.1) ,OTU(@c3e12f53@.2) ] ,XIC(@e392d01d@.Prove.Process.Sequencing.Phase.Active) [OTL(@c3e12f53@.0) ,OTU(@c3e12f53@.1) ,OTU(@c3e12f53@.2) ] ,XIC(@e392d01d@.Prove.Process.Sequencing.Phase.CountingPast1stSwitch) [OTU(@c3e12f53@.0) ,OTL(@c3e12f53@.1) ,OTU(@c3e12f53@.2) ] ,XIC(@e392d01d@.Prove.Process.Sequencing.Phase.Past2ndSwitchFwdLeg) [OTL(@c3e12f53@.0) ,OTL(@c3e12f53@.1) ,OTU(@c3e12f53@.2) ] ,XIC(@e392d01d@.Prove.Process.Sequencing.Phase.Past1stSwithRetLeg) [OTU(@c3e12f53@.0) ,OTU(@c3e12f53@.1) ,OTL(@c3e12f53@.2) ] ,XIC(@e392d01d@.Prove.Process.Sequencing.Phase.RunComplete) [OTL(@c3e12f53@.0) ,OTU(@c3e12f53@.1) ,OTL(@c3e12f53@.2) ] ,NEQ(@c3e12f53@,1) NEQ(@c3e12f53@,2) NEQ(@c3e12f53@,3) NEQ(@c3e12f53@,4) NEQ(@c3e12f53@,5) [OTL(@e392d01d@.Prove.Process.Sequencing.Phase.NotSelected) ,OTU(@e392d01d@.Prove.Process.Sequencing.Phase.Active) ,OTU(@e392d01d@.Prove.Process.Sequencing.Phase.CountingPast1stSwitch) ,OTU(@e392d01d@.Prove.Process.Sequencing.Phase.Past2ndSwitchFwdLeg) ,OTU(@e392d01d@.Prove.Process.Sequencing.Phase.Past1stSwithRetLeg) ,OTU(@e392d01d@.Prove.Process.Sequencing.Phase.RunComplete) ,MOV(0,@c3e12f53@) ] ,XIC(@e392d01d@.Prove.Process.Sequencing.BallPositionReady) OTL(@c3e12f53@.8) ,XIC(@e392d01d@.Prove.Process.Sequencing.BallPositionSealed) OTL(@c3e12f53@.9) ,XIC(@e392d01d@.Prove.Process.Sequencing.BallPositionReadyBwdLeg) OTL(@c3e12f53@.10) ,XIC(@e392d01d@.Prove.Process.Sequencing.BallPositionSealedBwdLeg) OTL(@c3e12f53@.11) ,MOV(16#7C00,@e392d01d@.Util.Buffer.Prove[0]) ,MOV(@c3e12f53@,@e392d01d@.Util.Buffer.Prove[1]) ,COP(@e392d01d@.Prove.Process.Temperature,@e392d01d@.Util.Buffer.Prove[4],2) ,COP(@e392d01d@.Prove.Process.OutletTemperature,@e392d01d@.Util.Buffer.Prove[6],2) ,COP(@e392d01d@.Prove.Process.SwitchBarTemperature,@e392d01d@.Util.Buffer.Prove[8],2) ,COP(@e392d01d@.Prove.Process.Pressure,@e392d01d@.Util.Buffer.Prove[10],2) ,COP(@e392d01d@.Prove.Process.OutletPressure,@e392d01d@.Util.Buffer.Prove[12],2) ,COP(@e392d01d@.Prove.Process.ProverDensity,@e392d01d@.Util.Buffer.Prove[14],2) ,MOV(0,@1f384e10@) ,XIC(@e392d01d@.Prove.Signals.EnableProve) OTL(@1f384e10@.1) ,XIC(@e392d01d@.Prove.Signals.AcceptProve) OTL(@1f384e10@.2) ,XIC(@e392d01d@.Prove.Signals.RejectProve) OTL(@1f384e10@.3) ,XIC(@e392d01d@.Prove.Signals.RunStart) OTL(@1f384e10@.4) ,XIC(@e392d01d@.Prove.Signals.RunComplete) OTL(@1f384e10@.5) ,XIC(@e392d01d@.Prove.Signals.RunCancel) OTL(@1f384e10@.6) ,XIC(@e392d01d@.Prove.Signals.RunDelete) OTL(@1f384e10@.7) ,XIC(@e392d01d@.Prove.Signals.PassComplete) OTL(@1f384e10@.9) ,XIC(@e392d01d@.Prove.Signals.PauseProve) OTL(@1f384e10@.12) ,XIC(@e392d01d@.Prove.Signals.AbortProve) OTL(@1f384e10@.14) ,MOV(@1f384e10@,@e392d01d@.Util.Buffer.Prove[16]) ,[MOV(0,@7618916a@) ,XIC(@e392d01d@.Prove.Config.Enable.AutoAcceptProve) OTL(@7618916a@.0) ,XIC(@e392d01d@.Prove.Config.Enable.AutoContinueProve) OTL(@7618916a@.1) ,XIC(@e392d01d@.Prove.Config.Accept.ApplyMFChangeAllStreams) OTL(@7618916a@.13) ,XIC(@e392d01d@.Prove.Config.Accept.ApplyMFChangeCurve) OTL(@7618916a@.14) ,XIC(@e392d01d@.Prove.Config.Accept.ApplyNewMF) OTL(@7618916a@.15) ,MOV(@7618916a@,@e392d01d@.Util.Buffer.Prove[17]) ,MOV(@e392d01d@.Prove.Config.Enable.MeterNumber,@e392d01d@.Util.Buffer.Prove[18]) ,MOV(@e392d01d@.Prove.Config.Accept.RequestedInterpolationPoint,@e392d01d@.Util.Buffer.Prove[21]) ] ,[COP(@e392d01d@.Prove.PulseCounts.Meter,@e392d01d@.Util.Buffer.Prove[22],2) ,COP(@e392d01d@.Prove.PulseCounts.MasterMeter,@e392d01d@.Util.Buffer.Prove[24],2) ] ];
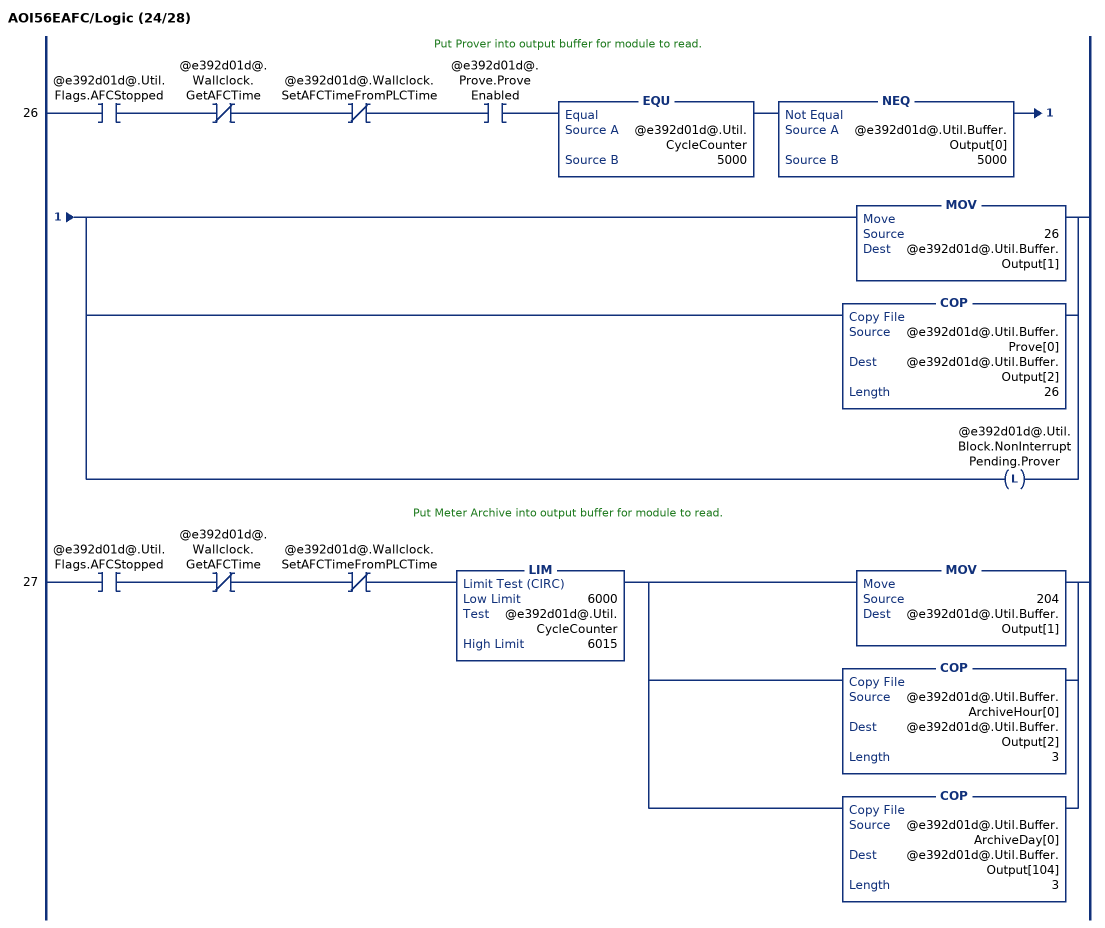
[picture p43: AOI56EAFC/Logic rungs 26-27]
   // Put Prover into output buffer for module to read.
   26: XIC(@e392d01d@.Util.Flags.AFCStopped)XIO(@e392d01d@.Wallclock.GetAFCTime)XIO(@e392d01d@.Wallclock.SetAFCTimeFromPLCTime)XIC(@e392d01d@.Prove.ProveEnabled)EQU(@e392d01d@.Util.CycleCounter,5000)NEQ(@e392d01d@.Util.Buffer.Output[0],5000)[MOV(26,@e392d01d@.Util.Buffer.Output[1]) ,COP(@e392d01d@.Util.Buffer.Prove[0],@e392d01d@.Util.Buffer.Output[2],26) ,OTL(@e392d01d@.Util.Block.NonInterruptPending.Prover) ];
   // Put Meter Archive into output buffer for module to read.
   27: XIC(@e392d01d@.Util.Flags.AFCStopped)XIO(@e392d01d@.Wallclock.GetAFCTime)XIO(@e392d01d@.Wallclock.SetAFCTimeFromPLCTime)LIM(6000,@e392d01d@.Util.CycleCounter,6015)[MOV(204,@e392d01d@.Util.Buffer.Output[1]) ,COP(@e392d01d@.Util.Buffer.ArchiveHour[0],@e392d01d@.Util.Buffer.Output[2],3) ,COP(@e392d01d@.Util.Buffer.ArchiveDay[0],@e392d01d@.Util.Buffer.Output[104],3) ];
